FUNCTION "FC_POWER_SAVING_MODE" : VOID
TITLE =POWER SAVING MODE
{ S7_language := '9(1) Angielski (Stany Zjednoczone)  21.09.2015  11:42:42' }
VERSION : 0.1


VAR_TEMP
  CDT : DATE_AND_TIME ;
  READ_CLOCK_RET_VAL : INT ;
  ACT_TIME : TIME_OF_DAY ;
  ACT_TIME_H : INT ;
  ACT_TIME_M : INT ;
  ACT_TIME_S : INT ;
  SW_WD1_ASU_STOP_HEATING : REAL ;
  SW_WD1_ASU_STOP_COOLING : REAL ;
  SW_WD2_ASU_STOP_HEATING : REAL ;
  SW_WD2_ASU_STOP_COOLING : REAL ;
END_VAR
BEGIN
NETWORK
TITLE =READING ACTUAL TIME FROM PLC
//********************************************************************************
//
//                         AUTOMATIC SETPOINTS UPDATE
//
//********************************************************************************
//
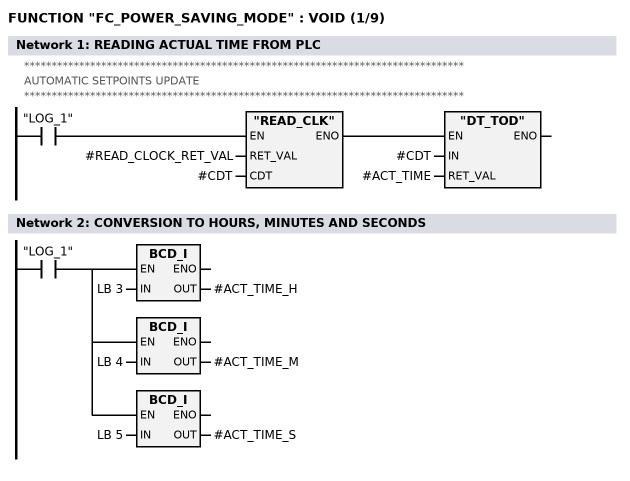
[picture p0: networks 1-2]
      U(    ;
      U     "LOG_1";
      SPBNB _001;
      CALL "READ_CLK" (
           RET_VAL                  := #READ_CLOCK_RET_VAL,
           CDT                      := #CDT);
_001: U     BIE;
      )     ;
      SPBNB _002;
      CALL "DT_TOD" (
           IN                       := #CDT,
           RET_VAL                  := #ACT_TIME);
_002: NOP   0;
NETWORK
TITLE =CONVERSION TO HOURS, MINUTES AND SECONDS

      U     "LOG_1";
      =     L     36.0;
      U     L     36.0;
      SPBNB _003;
      L     LB     3;
      BTI   ;
      T     #ACT_TIME_H;
_003: NOP   0;
      U     L     36.0;
      SPBNB _004;
      L     LB     4;
      BTI   ;
      T     #ACT_TIME_M;
_004: NOP   0;
      U     L     36.0;
      SPBNB _005;
      L     LB     5;
      BTI   ;
      T     #ACT_TIME_S;
_005: NOP   0;
NETWORK
TITLE =LIMIT TIME SET BY OPERATOR
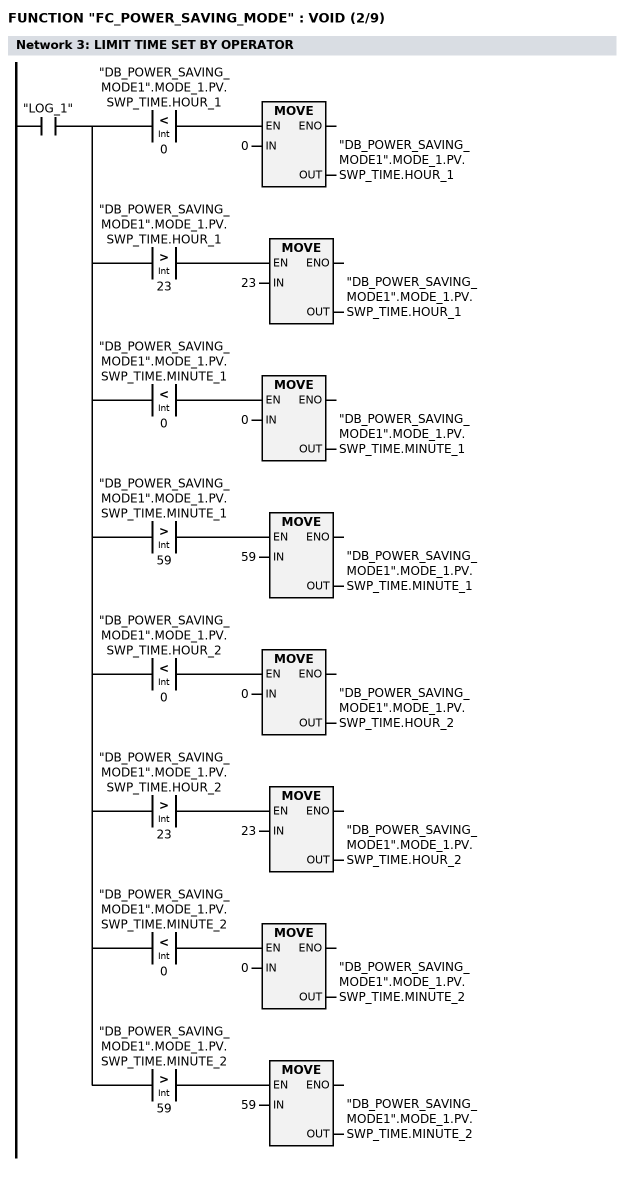
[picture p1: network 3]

      U     "LOG_1";
      =     L     36.0;
      U     L     36.0;
      U(    ;
      L     "DB_POWER_SAVING_MODE1".MODE_1.PV.SWP_TIME.HOUR_1;
      L     0;
      <I    ;
      )     ;
      SPBNB _006;
      L     0;
      T     "DB_POWER_SAVING_MODE1".MODE_1.PV.SWP_TIME.HOUR_1;
_006: NOP   0;
      U     L     36.0;
      U(    ;
      L     "DB_POWER_SAVING_MODE1".MODE_1.PV.SWP_TIME.HOUR_1;
      L     23;
      >I    ;
      )     ;
      SPBNB _007;
      L     23;
      T     "DB_POWER_SAVING_MODE1".MODE_1.PV.SWP_TIME.HOUR_1;
_007: NOP   0;
      U     L     36.0;
      U(    ;
      L     "DB_POWER_SAVING_MODE1".MODE_1.PV.SWP_TIME.MINUTE_1;
      L     0;
      <I    ;
      )     ;
      SPBNB _008;
      L     0;
      T     "DB_POWER_SAVING_MODE1".MODE_1.PV.SWP_TIME.MINUTE_1;
_008: NOP   0;
      U     L     36.0;
      U(    ;
      L     "DB_POWER_SAVING_MODE1".MODE_1.PV.SWP_TIME.MINUTE_1;
      L     59;
      >I    ;
      )     ;
      SPBNB _009;
      L     59;
      T     "DB_POWER_SAVING_MODE1".MODE_1.PV.SWP_TIME.MINUTE_1;
_009: NOP   0;
      U     L     36.0;
      U(    ;
      L     "DB_POWER_SAVING_MODE1".MODE_1.PV.SWP_TIME.HOUR_2;
      L     0;
      <I    ;
      )     ;
      SPBNB _00a;
      L     0;
      T     "DB_POWER_SAVING_MODE1".MODE_1.PV.SWP_TIME.HOUR_2;
_00a: NOP   0;
      U     L     36.0;
      U(    ;
      L     "DB_POWER_SAVING_MODE1".MODE_1.PV.SWP_TIME.HOUR_2;
      L     23;
      >I    ;
      )     ;
      SPBNB _00b;
      L     23;
      T     "DB_POWER_SAVING_MODE1".MODE_1.PV.SWP_TIME.HOUR_2;
_00b: NOP   0;
      U     L     36.0;
      U(    ;
      L     "DB_POWER_SAVING_MODE1".MODE_1.PV.SWP_TIME.MINUTE_2;
      L     0;
      <I    ;
      )     ;
      SPBNB _00c;
      L     0;
      T     "DB_POWER_SAVING_MODE1".MODE_1.PV.SWP_TIME.MINUTE_2;
_00c: NOP   0;
      U     L     36.0;
      U(    ;
      L     "DB_POWER_SAVING_MODE1".MODE_1.PV.SWP_TIME.MINUTE_2;
      L     59;
      >I    ;
      )     ;
      SPBNB _00d;
      L     59;
      T     "DB_POWER_SAVING_MODE1".MODE_1.PV.SWP_TIME.MINUTE_2;
_00d: NOP   0;
NETWORK
TITLE =CHANGE SETPOINTS TWO TIMES PER DAY ACCORDING TO TIME SET
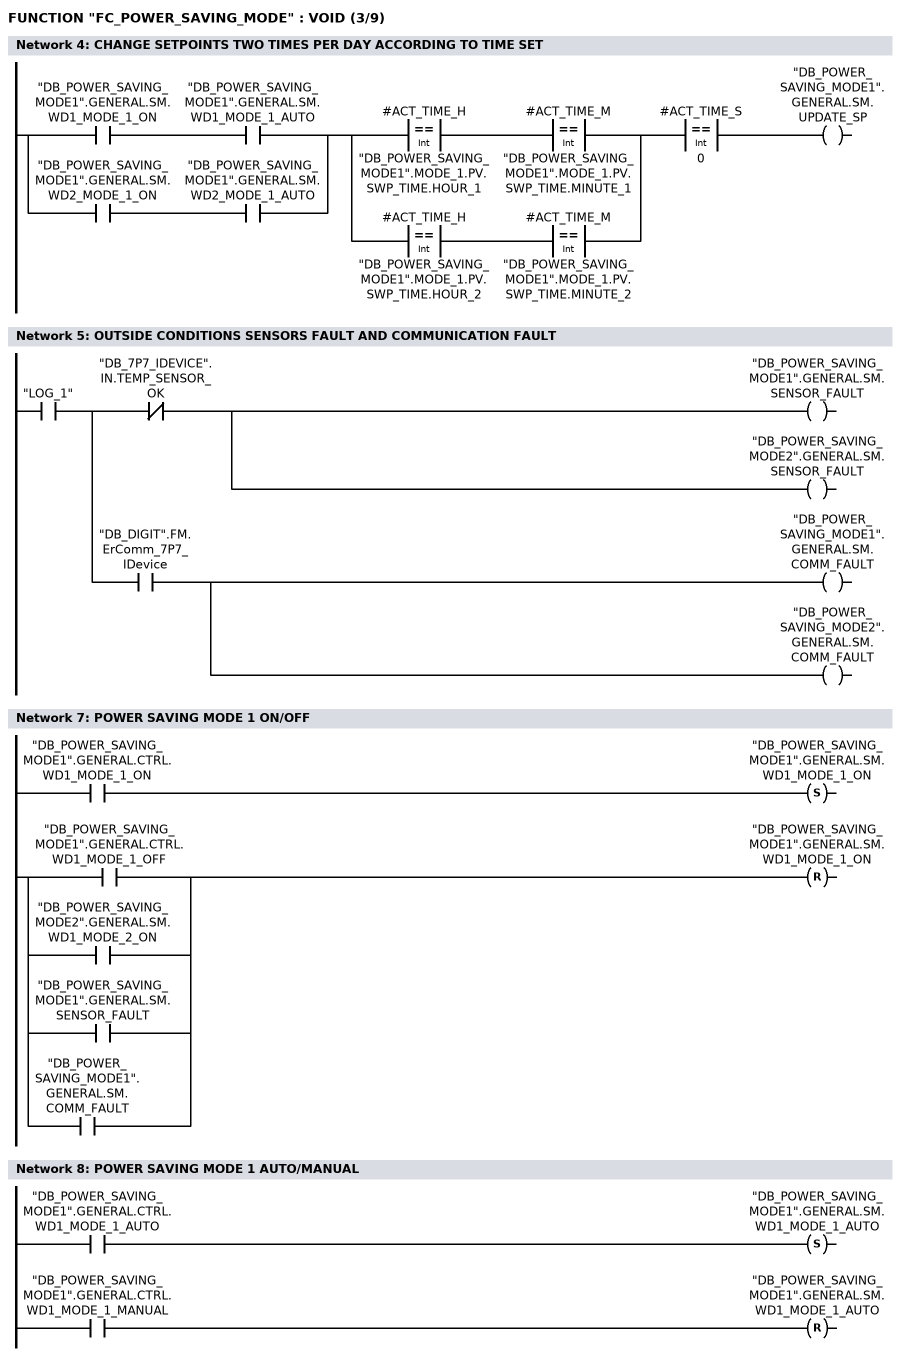
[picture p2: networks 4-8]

      U(    ;
      U     "DB_POWER_SAVING_MODE1".GENERAL.SM.WD1_MODE_1_ON;
      U     "DB_POWER_SAVING_MODE1".GENERAL.SM.WD1_MODE_1_AUTO;
      O     ;
      U     "DB_POWER_SAVING_MODE1".GENERAL.SM.WD2_MODE_1_ON;
      U     "DB_POWER_SAVING_MODE1".GENERAL.SM.WD2_MODE_1_AUTO;
      )     ;
      U(    ;
      U(    ;
      L     #ACT_TIME_H;
      L     "DB_POWER_SAVING_MODE1".MODE_1.PV.SWP_TIME.HOUR_1;
      ==I   ;
      )     ;
      U(    ;
      L     #ACT_TIME_M;
      L     "DB_POWER_SAVING_MODE1".MODE_1.PV.SWP_TIME.MINUTE_1;
      ==I   ;
      )     ;
      O     ;
      U(    ;
      L     #ACT_TIME_H;
      L     "DB_POWER_SAVING_MODE1".MODE_1.PV.SWP_TIME.HOUR_2;
      ==I   ;
      )     ;
      U(    ;
      L     #ACT_TIME_M;
      L     "DB_POWER_SAVING_MODE1".MODE_1.PV.SWP_TIME.MINUTE_2;
      ==I   ;
      )     ;
      )     ;
      U(    ;
      L     #ACT_TIME_S;
      L     0;
      ==I   ;
      )     ;
      =     "DB_POWER_SAVING_MODE1".GENERAL.SM.UPDATE_SP;
NETWORK
TITLE =OUTSIDE CONDITIONS SENSORS FAULT AND COMMUNICATION FAULT

      U     "LOG_1";
      =     L     36.0;
      U     L     36.0;
      UN    "DB_7P7_IDEVICE".IN.TEMP_SENSOR_OK;
      =     "DB_POWER_SAVING_MODE1".GENERAL.SM.SENSOR_FAULT;
      =     "DB_POWER_SAVING_MODE2".GENERAL.SM.SENSOR_FAULT;
      U     L     36.0;
      U     "DB_DIGIT".FM.ErComm_7P7_IDevice;
      =     "DB_POWER_SAVING_MODE1".GENERAL.SM.COMM_FAULT;
      =     "DB_POWER_SAVING_MODE2".GENERAL.SM.COMM_FAULT;
NETWORK
TITLE =********* WORKDECK'S 1 ECO MODE 1 **************
//********************************************************************************
//
//                     WORKDECK'S 1 POWER SAVING MODE 1
//
//********************************************************************************
//
NETWORK
TITLE =POWER SAVING MODE 1 ON/OFF

      U     "DB_POWER_SAVING_MODE1".GENERAL.CTRL.WD1_MODE_1_ON;
      S     "DB_POWER_SAVING_MODE1".GENERAL.SM.WD1_MODE_1_ON;
      U(    ;
      O     "DB_POWER_SAVING_MODE1".GENERAL.CTRL.WD1_MODE_1_OFF;
      O     "DB_POWER_SAVING_MODE2".GENERAL.SM.WD1_MODE_2_ON;
      O     "DB_POWER_SAVING_MODE1".GENERAL.SM.SENSOR_FAULT;
      O     "DB_POWER_SAVING_MODE1".GENERAL.SM.COMM_FAULT;
      )     ;
      R     "DB_POWER_SAVING_MODE1".GENERAL.SM.WD1_MODE_1_ON;
      NOP   0;
NETWORK
TITLE =POWER SAVING MODE 1 AUTO/MANUAL

      U     "DB_POWER_SAVING_MODE1".GENERAL.CTRL.WD1_MODE_1_AUTO;
      S     "DB_POWER_SAVING_MODE1".GENERAL.SM.WD1_MODE_1_AUTO;
      U     "DB_POWER_SAVING_MODE1".GENERAL.CTRL.WD1_MODE_1_MANUAL;
      R     "DB_POWER_SAVING_MODE1".GENERAL.SM.WD1_MODE_1_AUTO;
      NOP   0;
NETWORK
TITLE =
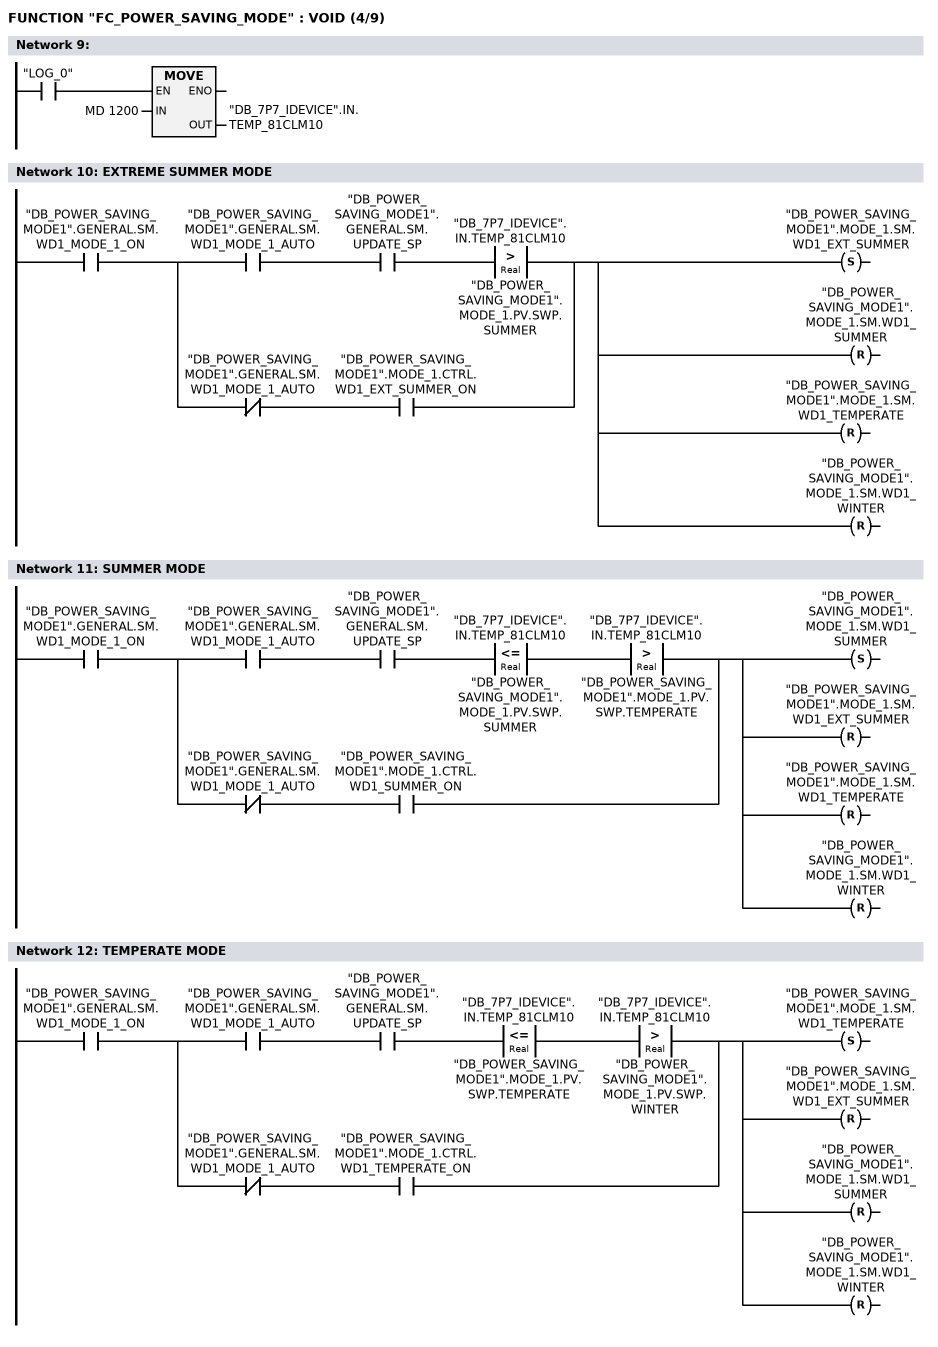
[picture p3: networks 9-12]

      U     "LOG_0";
      SPBNB _00e;
      L     MD  1200;
      T     "DB_7P7_IDEVICE".IN.TEMP_81CLM10;
_00e: NOP   0;
NETWORK
TITLE =EXTREME SUMMER MODE

      U     "DB_POWER_SAVING_MODE1".GENERAL.SM.WD1_MODE_1_ON;
      U(    ;
      U     "DB_POWER_SAVING_MODE1".GENERAL.SM.WD1_MODE_1_AUTO;
      U     "DB_POWER_SAVING_MODE1".GENERAL.SM.UPDATE_SP;
      U(    ;
      L     "DB_7P7_IDEVICE".IN.TEMP_81CLM10;
      L     "DB_POWER_SAVING_MODE1".MODE_1.PV.SWP.SUMMER;
      >R    ;
      )     ;
      O     ;
      UN    "DB_POWER_SAVING_MODE1".GENERAL.SM.WD1_MODE_1_AUTO;
      U     "DB_POWER_SAVING_MODE1".MODE_1.CTRL.WD1_EXT_SUMMER_ON;
      )     ;
      S     "DB_POWER_SAVING_MODE1".MODE_1.SM.WD1_EXT_SUMMER;
      R     "DB_POWER_SAVING_MODE1".MODE_1.SM.WD1_SUMMER;
      R     "DB_POWER_SAVING_MODE1".MODE_1.SM.WD1_TEMPERATE;
      R     "DB_POWER_SAVING_MODE1".MODE_1.SM.WD1_WINTER;
NETWORK
TITLE =SUMMER MODE

      U     "DB_POWER_SAVING_MODE1".GENERAL.SM.WD1_MODE_1_ON;
      U(    ;
      U     "DB_POWER_SAVING_MODE1".GENERAL.SM.WD1_MODE_1_AUTO;
      U     "DB_POWER_SAVING_MODE1".GENERAL.SM.UPDATE_SP;
      U(    ;
      L     "DB_7P7_IDEVICE".IN.TEMP_81CLM10;
      L     "DB_POWER_SAVING_MODE1".MODE_1.PV.SWP.SUMMER;
      <=R   ;
      )     ;
      U(    ;
      L     "DB_7P7_IDEVICE".IN.TEMP_81CLM10;
      L     "DB_POWER_SAVING_MODE1".MODE_1.PV.SWP.TEMPERATE;
      >R    ;
      )     ;
      O     ;
      UN    "DB_POWER_SAVING_MODE1".GENERAL.SM.WD1_MODE_1_AUTO;
      U     "DB_POWER_SAVING_MODE1".MODE_1.CTRL.WD1_SUMMER_ON;
      )     ;
      S     "DB_POWER_SAVING_MODE1".MODE_1.SM.WD1_SUMMER;
      R     "DB_POWER_SAVING_MODE1".MODE_1.SM.WD1_EXT_SUMMER;
      R     "DB_POWER_SAVING_MODE1".MODE_1.SM.WD1_TEMPERATE;
      R     "DB_POWER_SAVING_MODE1".MODE_1.SM.WD1_WINTER;
NETWORK
TITLE =TEMPERATE MODE

      U     "DB_POWER_SAVING_MODE1".GENERAL.SM.WD1_MODE_1_ON;
      U(    ;
      U     "DB_POWER_SAVING_MODE1".GENERAL.SM.WD1_MODE_1_AUTO;
      U     "DB_POWER_SAVING_MODE1".GENERAL.SM.UPDATE_SP;
      U(    ;
      L     "DB_7P7_IDEVICE".IN.TEMP_81CLM10;
      L     "DB_POWER_SAVING_MODE1".MODE_1.PV.SWP.TEMPERATE;
      <=R   ;
      )     ;
      U(    ;
      L     "DB_7P7_IDEVICE".IN.TEMP_81CLM10;
      L     "DB_POWER_SAVING_MODE1".MODE_1.PV.SWP.WINTER;
      >R    ;
      )     ;
      O     ;
      UN    "DB_POWER_SAVING_MODE1".GENERAL.SM.WD1_MODE_1_AUTO;
      U     "DB_POWER_SAVING_MODE1".MODE_1.CTRL.WD1_TEMPERATE_ON;
      )     ;
      S     "DB_POWER_SAVING_MODE1".MODE_1.SM.WD1_TEMPERATE;
      R     "DB_POWER_SAVING_MODE1".MODE_1.SM.WD1_EXT_SUMMER;
      R     "DB_POWER_SAVING_MODE1".MODE_1.SM.WD1_SUMMER;
      R     "DB_POWER_SAVING_MODE1".MODE_1.SM.WD1_WINTER;
NETWORK
TITLE =WINTER MODE
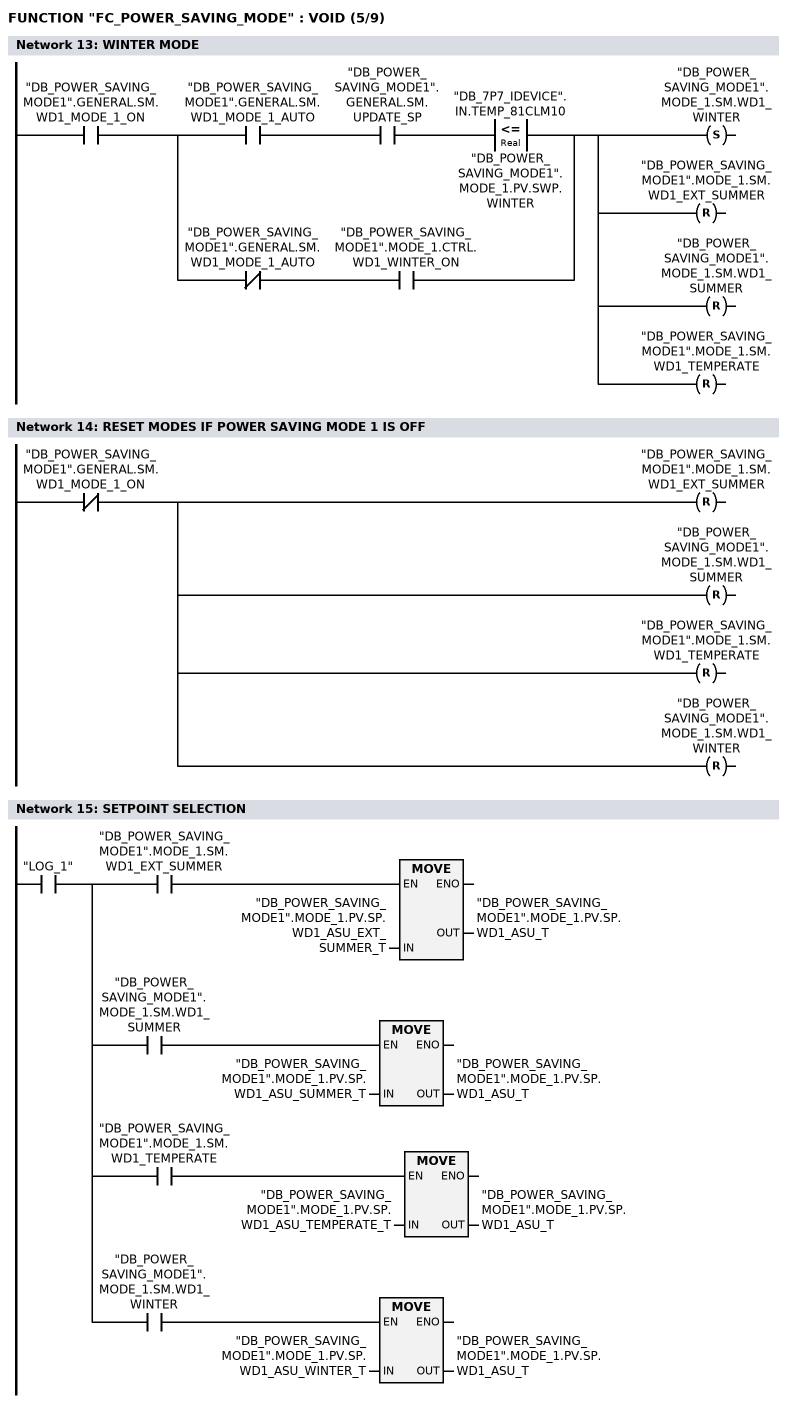
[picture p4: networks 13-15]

      U     "DB_POWER_SAVING_MODE1".GENERAL.SM.WD1_MODE_1_ON;
      U(    ;
      U     "DB_POWER_SAVING_MODE1".GENERAL.SM.WD1_MODE_1_AUTO;
      U     "DB_POWER_SAVING_MODE1".GENERAL.SM.UPDATE_SP;
      U(    ;
      L     "DB_7P7_IDEVICE".IN.TEMP_81CLM10;
      L     "DB_POWER_SAVING_MODE1".MODE_1.PV.SWP.WINTER;
      <=R   ;
      )     ;
      O     ;
      UN    "DB_POWER_SAVING_MODE1".GENERAL.SM.WD1_MODE_1_AUTO;
      U     "DB_POWER_SAVING_MODE1".MODE_1.CTRL.WD1_WINTER_ON;
      )     ;
      S     "DB_POWER_SAVING_MODE1".MODE_1.SM.WD1_WINTER;
      R     "DB_POWER_SAVING_MODE1".MODE_1.SM.WD1_EXT_SUMMER;
      R     "DB_POWER_SAVING_MODE1".MODE_1.SM.WD1_SUMMER;
      R     "DB_POWER_SAVING_MODE1".MODE_1.SM.WD1_TEMPERATE;
NETWORK
TITLE =RESET MODES IF POWER SAVING MODE 1 IS OFF

      UN    "DB_POWER_SAVING_MODE1".GENERAL.SM.WD1_MODE_1_ON;
      R     "DB_POWER_SAVING_MODE1".MODE_1.SM.WD1_EXT_SUMMER;
      R     "DB_POWER_SAVING_MODE1".MODE_1.SM.WD1_SUMMER;
      R     "DB_POWER_SAVING_MODE1".MODE_1.SM.WD1_TEMPERATE;
      R     "DB_POWER_SAVING_MODE1".MODE_1.SM.WD1_WINTER;
NETWORK
TITLE =SETPOINT SELECTION

      U     "LOG_1";
      =     L     36.0;
      U     L     36.0;
      U     "DB_POWER_SAVING_MODE1".MODE_1.SM.WD1_EXT_SUMMER;
      SPBNB _00f;
      L     "DB_POWER_SAVING_MODE1".MODE_1.PV.SP.WD1_ASU_EXT_SUMMER_T;
      T     "DB_POWER_SAVING_MODE1".MODE_1.PV.SP.WD1_ASU_T;
_00f: NOP   0;
      U     L     36.0;
      U     "DB_POWER_SAVING_MODE1".MODE_1.SM.WD1_SUMMER;
      SPBNB _010;
      L     "DB_POWER_SAVING_MODE1".MODE_1.PV.SP.WD1_ASU_SUMMER_T;
      T     "DB_POWER_SAVING_MODE1".MODE_1.PV.SP.WD1_ASU_T;
_010: NOP   0;
      U     L     36.0;
      U     "DB_POWER_SAVING_MODE1".MODE_1.SM.WD1_TEMPERATE;
      SPBNB _011;
      L     "DB_POWER_SAVING_MODE1".MODE_1.PV.SP.WD1_ASU_TEMPERATE_T;
      T     "DB_POWER_SAVING_MODE1".MODE_1.PV.SP.WD1_ASU_T;
_011: NOP   0;
      U     L     36.0;
      U     "DB_POWER_SAVING_MODE1".MODE_1.SM.WD1_WINTER;
      SPBNB _012;
      L     "DB_POWER_SAVING_MODE1".MODE_1.PV.SP.WD1_ASU_WINTER_T;
      T     "DB_POWER_SAVING_MODE1".MODE_1.PV.SP.WD1_ASU_T;
_012: NOP   0;
NETWORK
TITLE =DEFAULT MODE - TEMPERATE
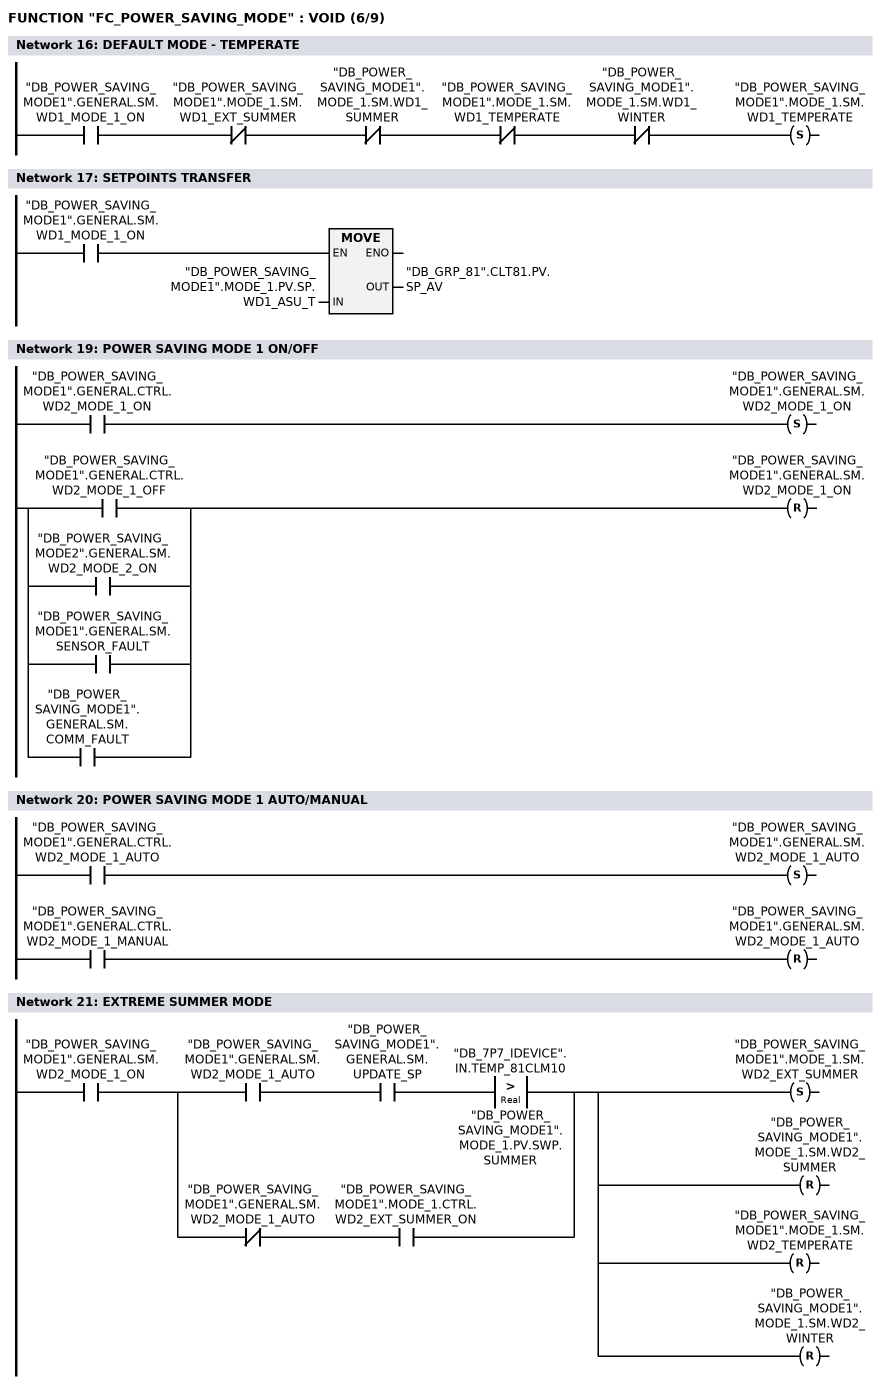
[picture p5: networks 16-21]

      U     "DB_POWER_SAVING_MODE1".GENERAL.SM.WD1_MODE_1_ON;
      UN    "DB_POWER_SAVING_MODE1".MODE_1.SM.WD1_EXT_SUMMER;
      UN    "DB_POWER_SAVING_MODE1".MODE_1.SM.WD1_SUMMER;
      UN    "DB_POWER_SAVING_MODE1".MODE_1.SM.WD1_TEMPERATE;
      UN    "DB_POWER_SAVING_MODE1".MODE_1.SM.WD1_WINTER;
      S     "DB_POWER_SAVING_MODE1".MODE_1.SM.WD1_TEMPERATE;
NETWORK
TITLE =SETPOINTS TRANSFER

      U     "DB_POWER_SAVING_MODE1".GENERAL.SM.WD1_MODE_1_ON;
      SPBNB _013;
      L     "DB_POWER_SAVING_MODE1".MODE_1.PV.SP.WD1_ASU_T;
      T     "DB_GRP_81".CLT81.PV.SP_AV;
_013: NOP   0;
NETWORK
TITLE =************ WORKDECK'S 2 ECO MODE 1 ***********
//********************************************************************************
//
//                        WORKDECK'S 2 POWER SAVING MODE 1
//
//********************************************************************************
//
NETWORK
TITLE =POWER SAVING MODE 1 ON/OFF

      U     "DB_POWER_SAVING_MODE1".GENERAL.CTRL.WD2_MODE_1_ON;
      S     "DB_POWER_SAVING_MODE1".GENERAL.SM.WD2_MODE_1_ON;
      U(    ;
      O     "DB_POWER_SAVING_MODE1".GENERAL.CTRL.WD2_MODE_1_OFF;
      O     "DB_POWER_SAVING_MODE2".GENERAL.SM.WD2_MODE_2_ON;
      O     "DB_POWER_SAVING_MODE1".GENERAL.SM.SENSOR_FAULT;
      O     "DB_POWER_SAVING_MODE1".GENERAL.SM.COMM_FAULT;
      )     ;
      R     "DB_POWER_SAVING_MODE1".GENERAL.SM.WD2_MODE_1_ON;
      NOP   0;
NETWORK
TITLE =POWER SAVING MODE 1 AUTO/MANUAL

      U     "DB_POWER_SAVING_MODE1".GENERAL.CTRL.WD2_MODE_1_AUTO;
      S     "DB_POWER_SAVING_MODE1".GENERAL.SM.WD2_MODE_1_AUTO;
      U     "DB_POWER_SAVING_MODE1".GENERAL.CTRL.WD2_MODE_1_MANUAL;
      R     "DB_POWER_SAVING_MODE1".GENERAL.SM.WD2_MODE_1_AUTO;
      NOP   0;
NETWORK
TITLE =EXTREME SUMMER MODE

      U     "DB_POWER_SAVING_MODE1".GENERAL.SM.WD2_MODE_1_ON;
      U(    ;
      U     "DB_POWER_SAVING_MODE1".GENERAL.SM.WD2_MODE_1_AUTO;
      U     "DB_POWER_SAVING_MODE1".GENERAL.SM.UPDATE_SP;
      U(    ;
      L     "DB_7P7_IDEVICE".IN.TEMP_81CLM10;
      L     "DB_POWER_SAVING_MODE1".MODE_1.PV.SWP.SUMMER;
      >R    ;
      )     ;
      O     ;
      UN    "DB_POWER_SAVING_MODE1".GENERAL.SM.WD2_MODE_1_AUTO;
      U     "DB_POWER_SAVING_MODE1".MODE_1.CTRL.WD2_EXT_SUMMER_ON;
      )     ;
      S     "DB_POWER_SAVING_MODE1".MODE_1.SM.WD2_EXT_SUMMER;
      R     "DB_POWER_SAVING_MODE1".MODE_1.SM.WD2_SUMMER;
      R     "DB_POWER_SAVING_MODE1".MODE_1.SM.WD2_TEMPERATE;
      R     "DB_POWER_SAVING_MODE1".MODE_1.SM.WD2_WINTER;
NETWORK
TITLE =SUMMER MODE
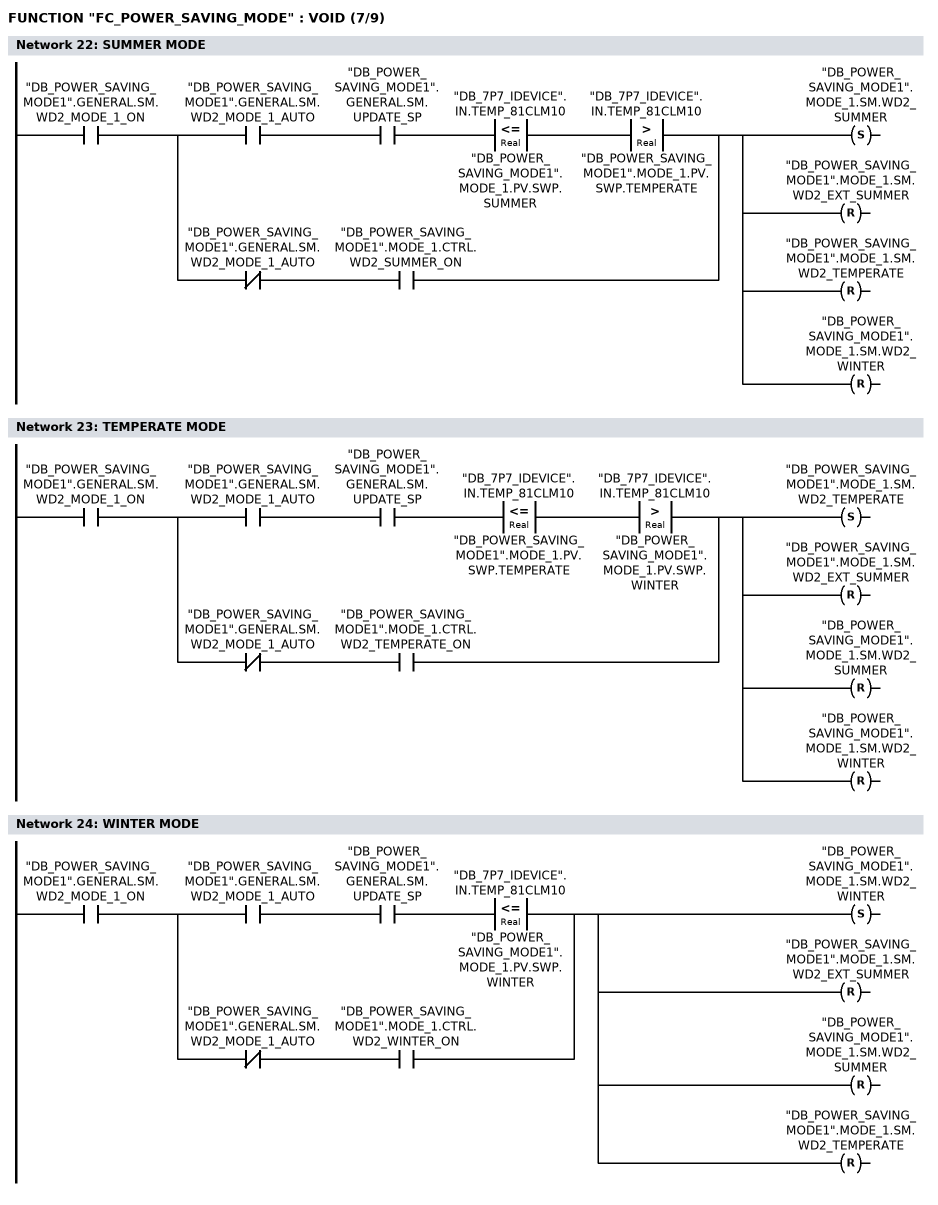
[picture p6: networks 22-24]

      U     "DB_POWER_SAVING_MODE1".GENERAL.SM.WD2_MODE_1_ON;
      U(    ;
      U     "DB_POWER_SAVING_MODE1".GENERAL.SM.WD2_MODE_1_AUTO;
      U     "DB_POWER_SAVING_MODE1".GENERAL.SM.UPDATE_SP;
      U(    ;
      L     "DB_7P7_IDEVICE".IN.TEMP_81CLM10;
      L     "DB_POWER_SAVING_MODE1".MODE_1.PV.SWP.SUMMER;
      <=R   ;
      )     ;
      U(    ;
      L     "DB_7P7_IDEVICE".IN.TEMP_81CLM10;
      L     "DB_POWER_SAVING_MODE1".MODE_1.PV.SWP.TEMPERATE;
      >R    ;
      )     ;
      O     ;
      UN    "DB_POWER_SAVING_MODE1".GENERAL.SM.WD2_MODE_1_AUTO;
      U     "DB_POWER_SAVING_MODE1".MODE_1.CTRL.WD2_SUMMER_ON;
      )     ;
      S     "DB_POWER_SAVING_MODE1".MODE_1.SM.WD2_SUMMER;
      R     "DB_POWER_SAVING_MODE1".MODE_1.SM.WD2_EXT_SUMMER;
      R     "DB_POWER_SAVING_MODE1".MODE_1.SM.WD2_TEMPERATE;
      R     "DB_POWER_SAVING_MODE1".MODE_1.SM.WD2_WINTER;
NETWORK
TITLE =TEMPERATE MODE

      U     "DB_POWER_SAVING_MODE1".GENERAL.SM.WD2_MODE_1_ON;
      U(    ;
      U     "DB_POWER_SAVING_MODE1".GENERAL.SM.WD2_MODE_1_AUTO;
      U     "DB_POWER_SAVING_MODE1".GENERAL.SM.UPDATE_SP;
      U(    ;
      L     "DB_7P7_IDEVICE".IN.TEMP_81CLM10;
      L     "DB_POWER_SAVING_MODE1".MODE_1.PV.SWP.TEMPERATE;
      <=R   ;
      )     ;
      U(    ;
      L     "DB_7P7_IDEVICE".IN.TEMP_81CLM10;
      L     "DB_POWER_SAVING_MODE1".MODE_1.PV.SWP.WINTER;
      >R    ;
      )     ;
      O     ;
      UN    "DB_POWER_SAVING_MODE1".GENERAL.SM.WD2_MODE_1_AUTO;
      U     "DB_POWER_SAVING_MODE1".MODE_1.CTRL.WD2_TEMPERATE_ON;
      )     ;
      S     "DB_POWER_SAVING_MODE1".MODE_1.SM.WD2_TEMPERATE;
      R     "DB_POWER_SAVING_MODE1".MODE_1.SM.WD2_EXT_SUMMER;
      R     "DB_POWER_SAVING_MODE1".MODE_1.SM.WD2_SUMMER;
      R     "DB_POWER_SAVING_MODE1".MODE_1.SM.WD2_WINTER;
NETWORK
TITLE =WINTER MODE

      U     "DB_POWER_SAVING_MODE1".GENERAL.SM.WD2_MODE_1_ON;
      U(    ;
      U     "DB_POWER_SAVING_MODE1".GENERAL.SM.WD2_MODE_1_AUTO;
      U     "DB_POWER_SAVING_MODE1".GENERAL.SM.UPDATE_SP;
      U(    ;
      L     "DB_7P7_IDEVICE".IN.TEMP_81CLM10;
      L     "DB_POWER_SAVING_MODE1".MODE_1.PV.SWP.WINTER;
      <=R   ;
      )     ;
      O     ;
      UN    "DB_POWER_SAVING_MODE1".GENERAL.SM.WD2_MODE_1_AUTO;
      U     "DB_POWER_SAVING_MODE1".MODE_1.CTRL.WD2_WINTER_ON;
      )     ;
      S     "DB_POWER_SAVING_MODE1".MODE_1.SM.WD2_WINTER;
      R     "DB_POWER_SAVING_MODE1".MODE_1.SM.WD2_EXT_SUMMER;
      R     "DB_POWER_SAVING_MODE1".MODE_1.SM.WD2_SUMMER;
      R     "DB_POWER_SAVING_MODE1".MODE_1.SM.WD2_TEMPERATE;
NETWORK
TITLE =RESET MODES IF POWER SAVING MODE 1 IS OFF
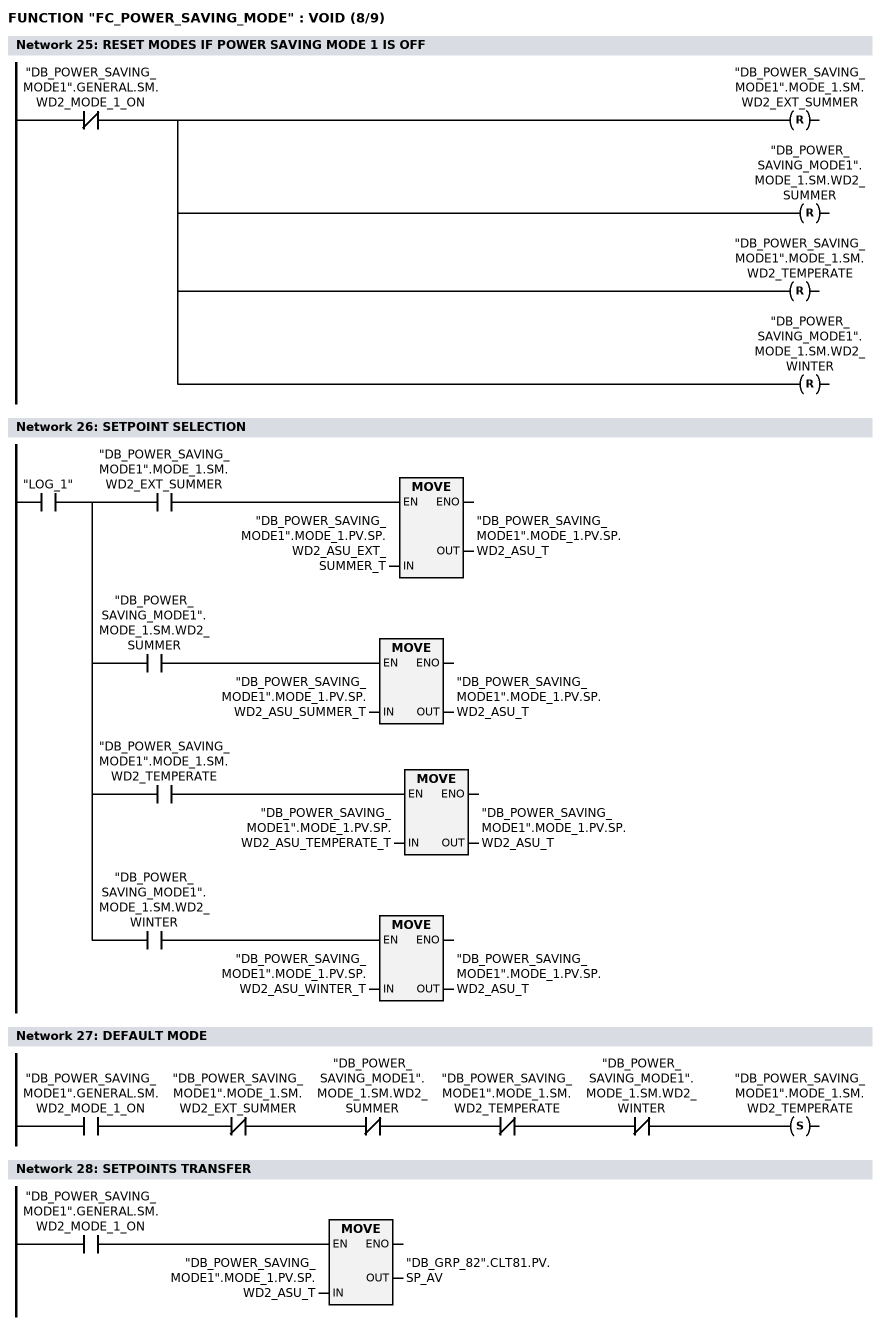
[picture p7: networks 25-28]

      UN    "DB_POWER_SAVING_MODE1".GENERAL.SM.WD2_MODE_1_ON;
      R     "DB_POWER_SAVING_MODE1".MODE_1.SM.WD2_EXT_SUMMER;
      R     "DB_POWER_SAVING_MODE1".MODE_1.SM.WD2_SUMMER;
      R     "DB_POWER_SAVING_MODE1".MODE_1.SM.WD2_TEMPERATE;
      R     "DB_POWER_SAVING_MODE1".MODE_1.SM.WD2_WINTER;
NETWORK
TITLE =SETPOINT SELECTION

      U     "LOG_1";
      =     L     36.0;
      U     L     36.0;
      U     "DB_POWER_SAVING_MODE1".MODE_1.SM.WD2_EXT_SUMMER;
      SPBNB _014;
      L     "DB_POWER_SAVING_MODE1".MODE_1.PV.SP.WD2_ASU_EXT_SUMMER_T;
      T     "DB_POWER_SAVING_MODE1".MODE_1.PV.SP.WD2_ASU_T;
_014: NOP   0;
      U     L     36.0;
      U     "DB_POWER_SAVING_MODE1".MODE_1.SM.WD2_SUMMER;
      SPBNB _015;
      L     "DB_POWER_SAVING_MODE1".MODE_1.PV.SP.WD2_ASU_SUMMER_T;
      T     "DB_POWER_SAVING_MODE1".MODE_1.PV.SP.WD2_ASU_T;
_015: NOP   0;
      U     L     36.0;
      U     "DB_POWER_SAVING_MODE1".MODE_1.SM.WD2_TEMPERATE;
      SPBNB _016;
      L     "DB_POWER_SAVING_MODE1".MODE_1.PV.SP.WD2_ASU_TEMPERATE_T;
      T     "DB_POWER_SAVING_MODE1".MODE_1.PV.SP.WD2_ASU_T;
_016: NOP   0;
      U     L     36.0;
      U     "DB_POWER_SAVING_MODE1".MODE_1.SM.WD2_WINTER;
      SPBNB _017;
      L     "DB_POWER_SAVING_MODE1".MODE_1.PV.SP.WD2_ASU_WINTER_T;
      T     "DB_POWER_SAVING_MODE1".MODE_1.PV.SP.WD2_ASU_T;
_017: NOP   0;
NETWORK
TITLE =DEFAULT MODE

      U     "DB_POWER_SAVING_MODE1".GENERAL.SM.WD2_MODE_1_ON;
      UN    "DB_POWER_SAVING_MODE1".MODE_1.SM.WD2_EXT_SUMMER;
      UN    "DB_POWER_SAVING_MODE1".MODE_1.SM.WD2_SUMMER;
      UN    "DB_POWER_SAVING_MODE1".MODE_1.SM.WD2_TEMPERATE;
      UN    "DB_POWER_SAVING_MODE1".MODE_1.SM.WD2_WINTER;
      S     "DB_POWER_SAVING_MODE1".MODE_1.SM.WD2_TEMPERATE;
NETWORK
TITLE =SETPOINTS TRANSFER

      U     "DB_POWER_SAVING_MODE1".GENERAL.SM.WD2_MODE_1_ON;
      SPBNB _018;
      L     "DB_POWER_SAVING_MODE1".MODE_1.PV.SP.WD2_ASU_T;
      T     "DB_GRP_82".CLT81.PV.SP_AV;
_018: NOP   0;
NETWORK
TITLE =************* WORKDECK'S 1/2 ECO MODE 2 ************
//********************************************************************************
//
//                     WORKDECK'S 1/2 POWER SAVING MODE 2
//
//********************************************************************************
//
NETWORK
TITLE =POWER SAVING MODE 2 WORKDECK'S 1 ON/OFF
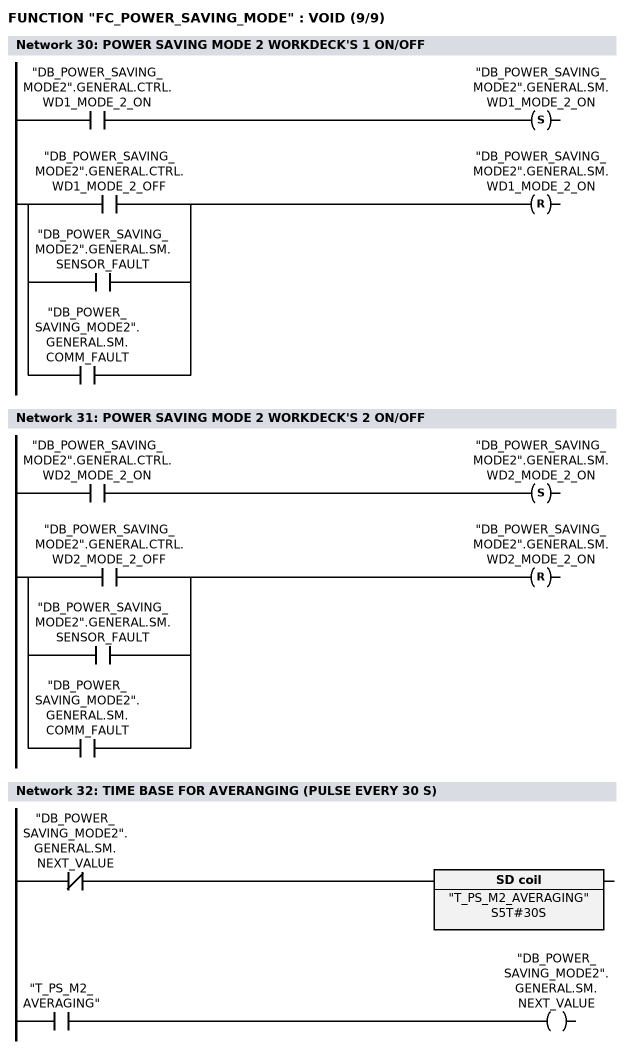
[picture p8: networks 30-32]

      U     "DB_POWER_SAVING_MODE2".GENERAL.CTRL.WD1_MODE_2_ON;
      S     "DB_POWER_SAVING_MODE2".GENERAL.SM.WD1_MODE_2_ON;
      U(    ;
      O     "DB_POWER_SAVING_MODE2".GENERAL.CTRL.WD1_MODE_2_OFF;
      O     "DB_POWER_SAVING_MODE2".GENERAL.SM.SENSOR_FAULT;
      O     "DB_POWER_SAVING_MODE2".GENERAL.SM.COMM_FAULT;
      )     ;
      R     "DB_POWER_SAVING_MODE2".GENERAL.SM.WD1_MODE_2_ON;
      NOP   0;
NETWORK
TITLE =POWER SAVING MODE 2 WORKDECK'S 2 ON/OFF

      U     "DB_POWER_SAVING_MODE2".GENERAL.CTRL.WD2_MODE_2_ON;
      S     "DB_POWER_SAVING_MODE2".GENERAL.SM.WD2_MODE_2_ON;
      U(    ;
      O     "DB_POWER_SAVING_MODE2".GENERAL.CTRL.WD2_MODE_2_OFF;
      O     "DB_POWER_SAVING_MODE2".GENERAL.SM.SENSOR_FAULT;
      O     "DB_POWER_SAVING_MODE2".GENERAL.SM.COMM_FAULT;
      )     ;
      R     "DB_POWER_SAVING_MODE2".GENERAL.SM.WD2_MODE_2_ON;
      NOP   0;
NETWORK
TITLE =TIME BASE FOR AVERANGING (PULSE EVERY 30 S)

      UN    "DB_POWER_SAVING_MODE2".GENERAL.SM.NEXT_VALUE;
      L     S5T#30S;
      SE    "T_PS_M2_AVERAGING";

      U     "T_PS_M2_AVERAGING";
      =     "DB_POWER_SAVING_MODE2".GENERAL.SM.NEXT_VALUE;

NETWORK
TITLE =10 MIN AVERAGE OF OUTSIDE TEMPERATURE

      UN    "DB_POWER_SAVING_MODE2".GENERAL.SM.SENSOR_FAULT;
      =     L     36.0;
      U     "DB_POWER_SAVING_MODE2".GENERAL.SM.NEXT_VALUE;
      =     L     36.1;
      BLD   103;
      U     L     36.0;
      SPBNB _019;
      CALL "FB_AVERAGING" , "DBI_81CLM10_TEMP_AVR" (
           IiNumberOfAddend         := 20,
           IrMeasuringValue         := "DB_7P7_IDEVICE".IN.TEMP_81CLM10,
           IxNewValueAvailable      := L     36.1);

_019: NOP   0;
      U     L     36.0;
      SPBNB _01a;
      L     "DBI_81CLM10_TEMP_AVR".QrAverageValue;
      T     "DB_POWER_SAVING_MODE2".GENERAL.PV.AVG_TEMP;
_01a: NOP   0;
NETWORK
TITLE =************** START ECO MODE 2 WORKDECK'S 1 *************

NETWORK
TITLE =WORKDECK'S 1 ASU OUTSIDE CONDITIONS
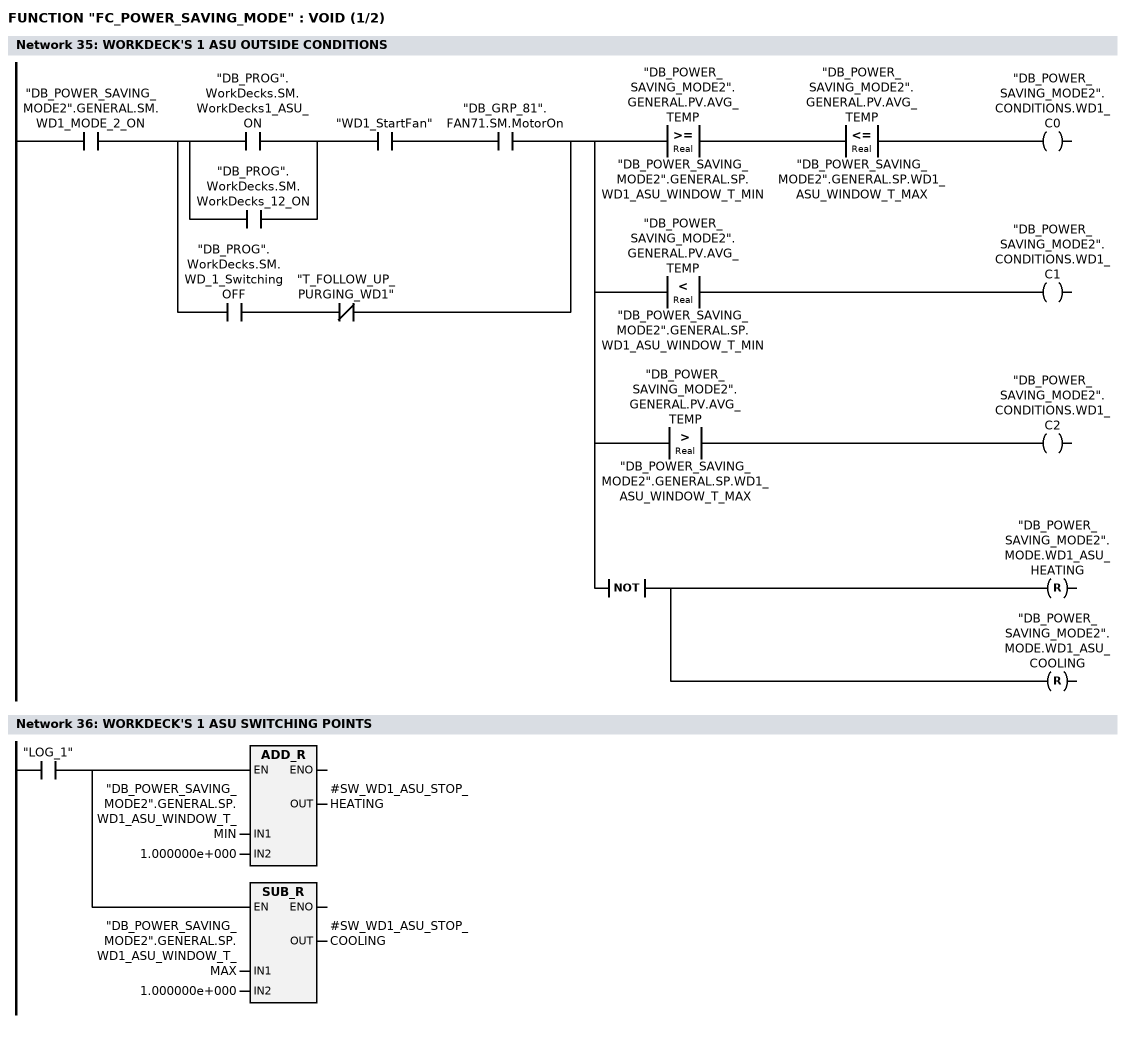
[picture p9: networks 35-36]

      U     "DB_POWER_SAVING_MODE2".GENERAL.SM.WD1_MODE_2_ON;
      U(    ;
      U(    ;
      O     "DB_PROG".WorkDecks.SM.WorkDecks1_ASU_ON;
      O     "DB_PROG".WorkDecks.SM.WorkDecks_12_ON;
      )     ;
      U     "WD1_StartFan";
      U     "DB_GRP_81".FAN71.SM.MotorOn;
      O     ;
      U     "DB_PROG".WorkDecks.SM.WD_1_SwitchingOFF;
      UN    "T_FOLLOW_UP_PURGING_WD1";
      )     ;
      =     L     36.0;
      U     L     36.0;
      U(    ;
      L     "DB_POWER_SAVING_MODE2".GENERAL.PV.AVG_TEMP;
      L     "DB_POWER_SAVING_MODE2".GENERAL.SP.WD1_ASU_WINDOW_T_MIN;
      >=R   ;
      )     ;
      U(    ;
      L     "DB_POWER_SAVING_MODE2".GENERAL.PV.AVG_TEMP;
      L     "DB_POWER_SAVING_MODE2".GENERAL.SP.WD1_ASU_WINDOW_T_MAX;
      <=R   ;
      )     ;
      =     "DB_POWER_SAVING_MODE2".CONDITIONS.WD1_C0;
      U     L     36.0;
      U(    ;
      L     "DB_POWER_SAVING_MODE2".GENERAL.PV.AVG_TEMP;
      L     "DB_POWER_SAVING_MODE2".GENERAL.SP.WD1_ASU_WINDOW_T_MIN;
      <R    ;
      )     ;
      =     "DB_POWER_SAVING_MODE2".CONDITIONS.WD1_C1;
      U     L     36.0;
      U(    ;
      L     "DB_POWER_SAVING_MODE2".GENERAL.PV.AVG_TEMP;
      L     "DB_POWER_SAVING_MODE2".GENERAL.SP.WD1_ASU_WINDOW_T_MAX;
      >R    ;
      )     ;
      =     "DB_POWER_SAVING_MODE2".CONDITIONS.WD1_C2;
      U     L     36.0;
      NOT   ;
      R     "DB_POWER_SAVING_MODE2".MODE.WD1_ASU_HEATING;
      R     "DB_POWER_SAVING_MODE2".MODE.WD1_ASU_COOLING;
NETWORK
TITLE =WORKDECK'S 1 ASU SWITCHING POINTS

      U     "LOG_1";
      =     L     36.0;
      U     L     36.0;
      SPBNB _01b;
      L     "DB_POWER_SAVING_MODE2".GENERAL.SP.WD1_ASU_WINDOW_T_MIN;
      L     1.000000e+000;
      +R    ;
      T     #SW_WD1_ASU_STOP_HEATING;
_01b: NOP   0;
      U     L     36.0;
      SPBNB _01c;
      L     "DB_POWER_SAVING_MODE2".GENERAL.SP.WD1_ASU_WINDOW_T_MAX;
      L     1.000000e+000;
      -R    ;
      T     #SW_WD1_ASU_STOP_COOLING;
_01c: NOP   0;
NETWORK
TITLE =WORKDECK'S 1 CONDIDITON 0
//OUTSIDE TEMPERATURE IN WINDOW
//
//HEATING OFF
//COOLING OFF
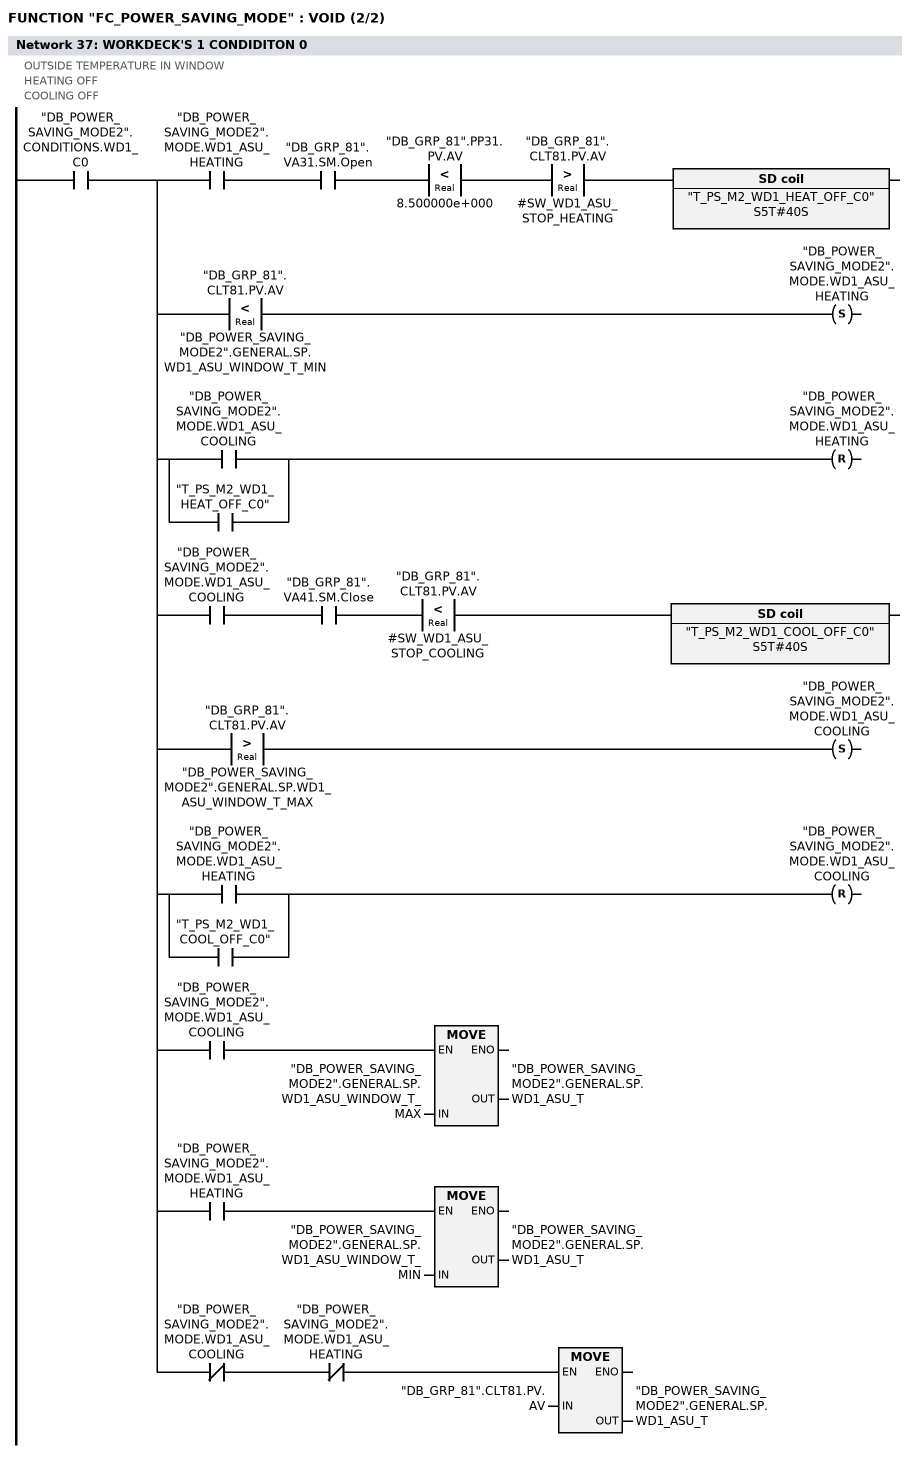
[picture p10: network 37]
      U     "DB_POWER_SAVING_MODE2".CONDITIONS.WD1_C0;
      =     L     36.0;
      U     L     36.0;
      U     "DB_POWER_SAVING_MODE2".MODE.WD1_ASU_HEATING;
      U     "DB_GRP_81".VA31.SM.Open;
      U(    ;
      L     "DB_GRP_81".PP31.PV.AV;
      L     8.500000e+000;
      <R    ;
      )     ;
      U(    ;
      L     "DB_GRP_81".CLT81.PV.AV;
      L     #SW_WD1_ASU_STOP_HEATING;
      >R    ;
      )     ;
      L     S5T#40S;
      SE    "T_PS_M2_WD1_HEAT_OFF_C0";
      NOP   0;
      NOP   0;
      NOP   0;
      NOP   0;
      U     L     36.0;
      U(    ;
      L     "DB_GRP_81".CLT81.PV.AV;
      L     "DB_POWER_SAVING_MODE2".GENERAL.SP.WD1_ASU_WINDOW_T_MIN;
      <R    ;
      )     ;
      S     "DB_POWER_SAVING_MODE2".MODE.WD1_ASU_HEATING;
      U     L     36.0;
      U(    ;
      O     "DB_POWER_SAVING_MODE2".MODE.WD1_ASU_COOLING;
      O     "T_PS_M2_WD1_HEAT_OFF_C0";
      )     ;
      R     "DB_POWER_SAVING_MODE2".MODE.WD1_ASU_HEATING;
      U     L     36.0;
      U     "DB_POWER_SAVING_MODE2".MODE.WD1_ASU_COOLING;
      U     "DB_GRP_81".VA41.SM.Close;
      U(    ;
      L     "DB_GRP_81".CLT81.PV.AV;
      L     #SW_WD1_ASU_STOP_COOLING;
      <R    ;
      )     ;
      L     S5T#40S;
      SE    "T_PS_M2_WD1_COOL_OFF_C0";
      NOP   0;
      NOP   0;
      NOP   0;
      NOP   0;
      U     L     36.0;
      U(    ;
      L     "DB_GRP_81".CLT81.PV.AV;
      L     "DB_POWER_SAVING_MODE2".GENERAL.SP.WD1_ASU_WINDOW_T_MAX;
      >R    ;
      )     ;
      S     "DB_POWER_SAVING_MODE2".MODE.WD1_ASU_COOLING;
      U     L     36.0;
      U(    ;
      O     "DB_POWER_SAVING_MODE2".MODE.WD1_ASU_HEATING;
      O     "T_PS_M2_WD1_COOL_OFF_C0";
      )     ;
      R     "DB_POWER_SAVING_MODE2".MODE.WD1_ASU_COOLING;
      U     L     36.0;
      U     "DB_POWER_SAVING_MODE2".MODE.WD1_ASU_COOLING;
      SPBNB _01d;
      L     "DB_POWER_SAVING_MODE2".GENERAL.SP.WD1_ASU_WINDOW_T_MAX;
      T     "DB_POWER_SAVING_MODE2".GENERAL.SP.WD1_ASU_T;
_01d: NOP   0;
      U     L     36.0;
      U     "DB_POWER_SAVING_MODE2".MODE.WD1_ASU_HEATING;
      SPBNB _01e;
      L     "DB_POWER_SAVING_MODE2".GENERAL.SP.WD1_ASU_WINDOW_T_MIN;
      T     "DB_POWER_SAVING_MODE2".GENERAL.SP.WD1_ASU_T;
_01e: NOP   0;
      U     L     36.0;
      UN    "DB_POWER_SAVING_MODE2".MODE.WD1_ASU_COOLING;
      UN    "DB_POWER_SAVING_MODE2".MODE.WD1_ASU_HEATING;
      SPBNB _01f;
      L     "DB_GRP_81".CLT81.PV.AV;
      T     "DB_POWER_SAVING_MODE2".GENERAL.SP.WD1_ASU_T;
_01f: NOP   0;
NETWORK
TITLE =WORKDECK'S 1 CONDITION 1
//OUTSIDE TEMPERATURE < T MIN
//
//HEATING ON
//COOLING OFF
//UNTIL WINDOW IS REACHED
//
//HEATING SP T MIN
      U     "DB_POWER_SAVING_MODE2".CONDITIONS.WD1_C1;
      =     L     36.0;
      U     L     36.0;
      BLD   102;
      R     "DB_POWER_SAVING_MODE2".MODE.WD1_ASU_COOLING;
      U     L     36.0;
      U(    ;
      L     "DB_GRP_81".CLT81.PV.AV;
      L     "DB_POWER_SAVING_MODE2".GENERAL.SP.WD1_ASU_WINDOW_T_MIN;
      <R    ;
      )     ;
      S     "DB_POWER_SAVING_MODE2".MODE.WD1_ASU_HEATING;
      U     L     36.0;
      U     "DB_POWER_SAVING_MODE2".MODE.WD1_ASU_HEATING;
      U     "DB_GRP_81".VA31.SM.Open;
      U(    ;
      L     "DB_GRP_81".PP31.PV.AV;
      L     8.000000e+000;
      <=R   ;
      )     ;
      U(    ;
      L     "DB_GRP_81".CLT81.PV.AV;
      L     #SW_WD1_ASU_STOP_HEATING;
      >R    ;
      )     ;
      L     S5T#40S;
      SE    "T_PS_M2_WD1_HEAT_OFF_C1";
      NOP   0;
      NOP   0;
      NOP   0;
      U     "T_PS_M2_WD1_HEAT_OFF_C1";
      R     "DB_POWER_SAVING_MODE2".MODE.WD1_ASU_HEATING;
      U     L     36.0;
      U     "DB_POWER_SAVING_MODE2".MODE.WD1_ASU_HEATING;
      SPBNB _020;
      L     "DB_POWER_SAVING_MODE2".GENERAL.SP.WD1_ASU_WINDOW_T_MIN;
      T     "DB_POWER_SAVING_MODE2".GENERAL.SP.WD1_ASU_T;
_020: NOP   0;
      U     L     36.0;
      UN    "DB_POWER_SAVING_MODE2".MODE.WD1_ASU_HEATING;
      SPBNB _021;
      L     "DB_GRP_81".CLT81.PV.AV;
      T     "DB_POWER_SAVING_MODE2".GENERAL.SP.WD1_ASU_T;
_021: NOP   0;
NETWORK
TITLE =WORKDECK'S 1 CONDITION 2
//OUTSIDE TEMPERATURE > T MAX
//
//HEATING OFF
//COOLING ON
//UNTIL WINDOW IS REACHED
//
//COOLING SP T MAX
      U     "DB_POWER_SAVING_MODE2".CONDITIONS.WD1_C2;
      =     L     36.0;
      U     L     36.0;
      U(    ;
      L     "DB_GRP_81".CLT81.PV.AV;
      L     "DB_POWER_SAVING_MODE2".GENERAL.SP.WD1_ASU_WINDOW_T_MAX;
      >R    ;
      )     ;
      S     "DB_POWER_SAVING_MODE2".MODE.WD1_ASU_COOLING;
      U     L     36.0;
      U     "DB_POWER_SAVING_MODE2".MODE.WD1_ASU_COOLING;
      U     "DB_GRP_81".VA41.SM.Close;
      U(    ;
      L     "DB_GRP_81".CLT81.PV.AV;
      L     #SW_WD1_ASU_STOP_COOLING;
      <R    ;
      )     ;
      L     S5T#1M;
      SE    "T_PS_M2_WD1_COOL_OFF_C2";
      NOP   0;
      NOP   0;
      NOP   0;
      U     "T_PS_M2_WD1_COOL_OFF_C2";
      R     "DB_POWER_SAVING_MODE2".MODE.WD1_ASU_COOLING;
      U     L     36.0;
      BLD   102;
      R     "DB_POWER_SAVING_MODE2".MODE.WD1_ASU_HEATING;
      U     L     36.0;
      U     "DB_POWER_SAVING_MODE2".MODE.WD1_ASU_COOLING;
      SPBNB _022;
      L     "DB_POWER_SAVING_MODE2".GENERAL.SP.WD1_ASU_WINDOW_T_MAX;
      T     "DB_POWER_SAVING_MODE2".GENERAL.SP.WD1_ASU_T;
_022: NOP   0;
      U     L     36.0;
      UN    "DB_POWER_SAVING_MODE2".MODE.WD1_ASU_COOLING;
      SPBNB _023;
      L     "DB_GRP_81".CLT81.PV.AV;
      T     "DB_POWER_SAVING_MODE2".GENERAL.SP.WD1_ASU_T;
_023: NOP   0;
NETWORK
TITLE =TRANSFER SETPOINTS FOR WORKDECK'S 1
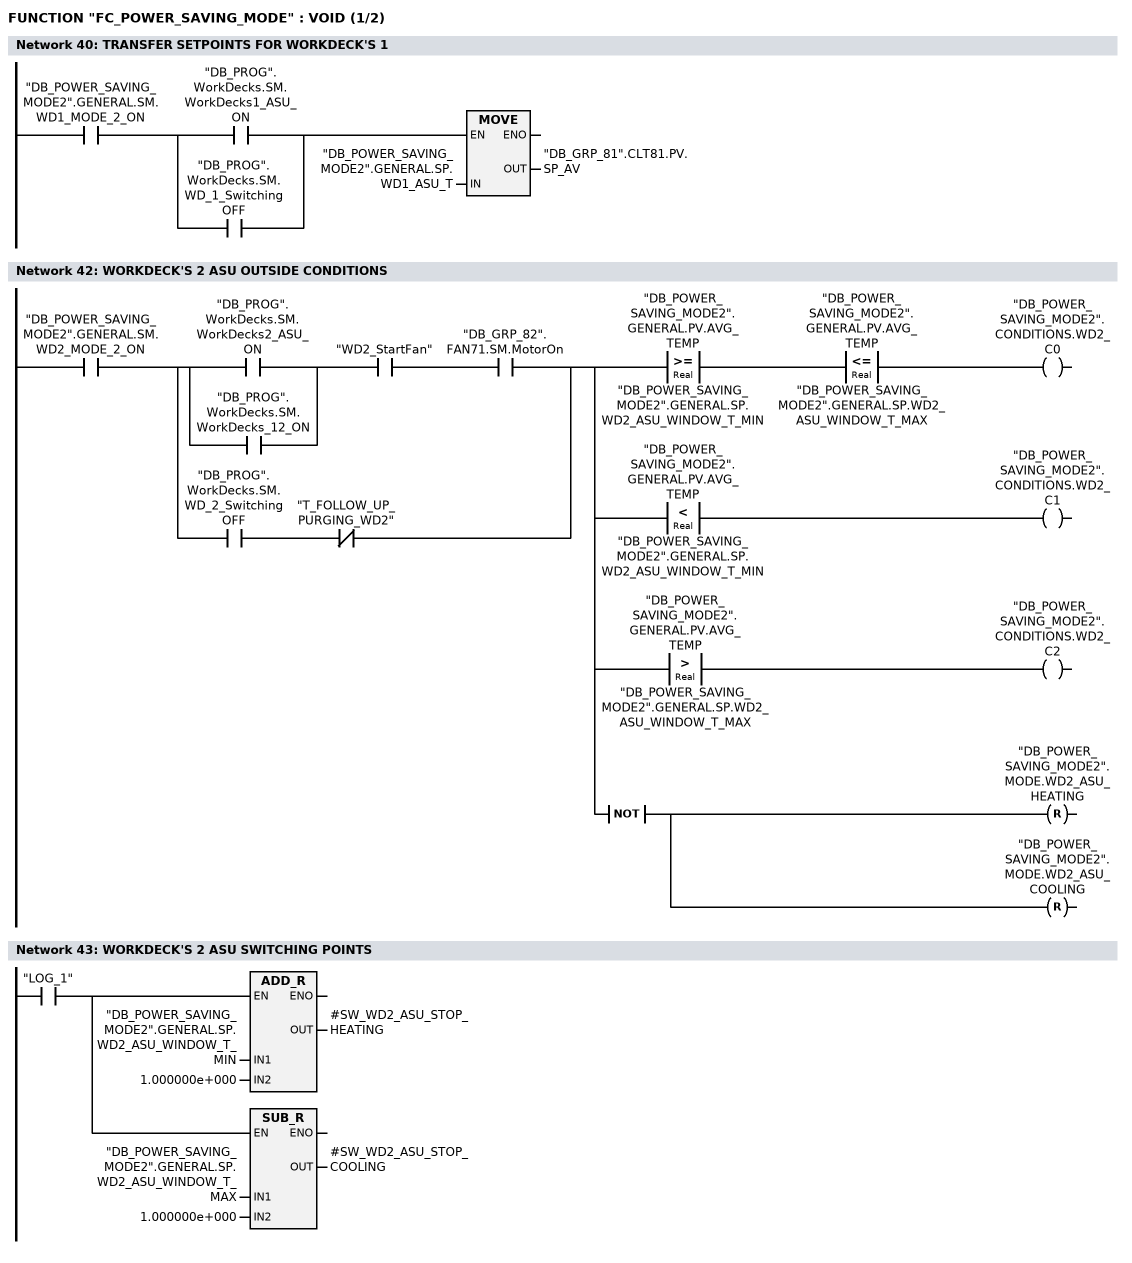
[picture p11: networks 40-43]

      U     "DB_POWER_SAVING_MODE2".GENERAL.SM.WD1_MODE_2_ON;
      U(    ;
      O     "DB_PROG".WorkDecks.SM.WorkDecks1_ASU_ON;
      O     "DB_PROG".WorkDecks.SM.WD_1_SwitchingOFF;
      )     ;
      SPBNB _024;
      L     "DB_POWER_SAVING_MODE2".GENERAL.SP.WD1_ASU_T;
      T     "DB_GRP_81".CLT81.PV.SP_AV;
_024: NOP   0;
NETWORK
TITLE =************** START ECO MODE 2 WORKDECK'S 2 *************

NETWORK
TITLE =WORKDECK'S 2 ASU OUTSIDE CONDITIONS

      U     "DB_POWER_SAVING_MODE2".GENERAL.SM.WD2_MODE_2_ON;
      U(    ;
      U(    ;
      O     "DB_PROG".WorkDecks.SM.WorkDecks2_ASU_ON;
      O     "DB_PROG".WorkDecks.SM.WorkDecks_12_ON;
      )     ;
      U     "WD2_StartFan";
      U     "DB_GRP_82".FAN71.SM.MotorOn;
      O     ;
      U     "DB_PROG".WorkDecks.SM.WD_2_SwitchingOFF;
      UN    "T_FOLLOW_UP_PURGING_WD2";
      )     ;
      =     L     36.0;
      U     L     36.0;
      U(    ;
      L     "DB_POWER_SAVING_MODE2".GENERAL.PV.AVG_TEMP;
      L     "DB_POWER_SAVING_MODE2".GENERAL.SP.WD2_ASU_WINDOW_T_MIN;
      >=R   ;
      )     ;
      U(    ;
      L     "DB_POWER_SAVING_MODE2".GENERAL.PV.AVG_TEMP;
      L     "DB_POWER_SAVING_MODE2".GENERAL.SP.WD2_ASU_WINDOW_T_MAX;
      <=R   ;
      )     ;
      =     "DB_POWER_SAVING_MODE2".CONDITIONS.WD2_C0;
      U     L     36.0;
      U(    ;
      L     "DB_POWER_SAVING_MODE2".GENERAL.PV.AVG_TEMP;
      L     "DB_POWER_SAVING_MODE2".GENERAL.SP.WD2_ASU_WINDOW_T_MIN;
      <R    ;
      )     ;
      =     "DB_POWER_SAVING_MODE2".CONDITIONS.WD2_C1;
      U     L     36.0;
      U(    ;
      L     "DB_POWER_SAVING_MODE2".GENERAL.PV.AVG_TEMP;
      L     "DB_POWER_SAVING_MODE2".GENERAL.SP.WD2_ASU_WINDOW_T_MAX;
      >R    ;
      )     ;
      =     "DB_POWER_SAVING_MODE2".CONDITIONS.WD2_C2;
      U     L     36.0;
      NOT   ;
      R     "DB_POWER_SAVING_MODE2".MODE.WD2_ASU_HEATING;
      R     "DB_POWER_SAVING_MODE2".MODE.WD2_ASU_COOLING;
NETWORK
TITLE =WORKDECK'S 2 ASU SWITCHING POINTS

      U     "LOG_1";
      =     L     36.0;
      U     L     36.0;
      SPBNB _025;
      L     "DB_POWER_SAVING_MODE2".GENERAL.SP.WD2_ASU_WINDOW_T_MIN;
      L     1.000000e+000;
      +R    ;
      T     #SW_WD2_ASU_STOP_HEATING;
_025: NOP   0;
      U     L     36.0;
      SPBNB _026;
      L     "DB_POWER_SAVING_MODE2".GENERAL.SP.WD2_ASU_WINDOW_T_MAX;
      L     1.000000e+000;
      -R    ;
      T     #SW_WD2_ASU_STOP_COOLING;
_026: NOP   0;
NETWORK
TITLE =WORKDECK'S 2 CONDIDITON 0
//OUTSIDE TEMPERATURE IN WINDOW
//
//HEATING OFF
//COOLING OFF
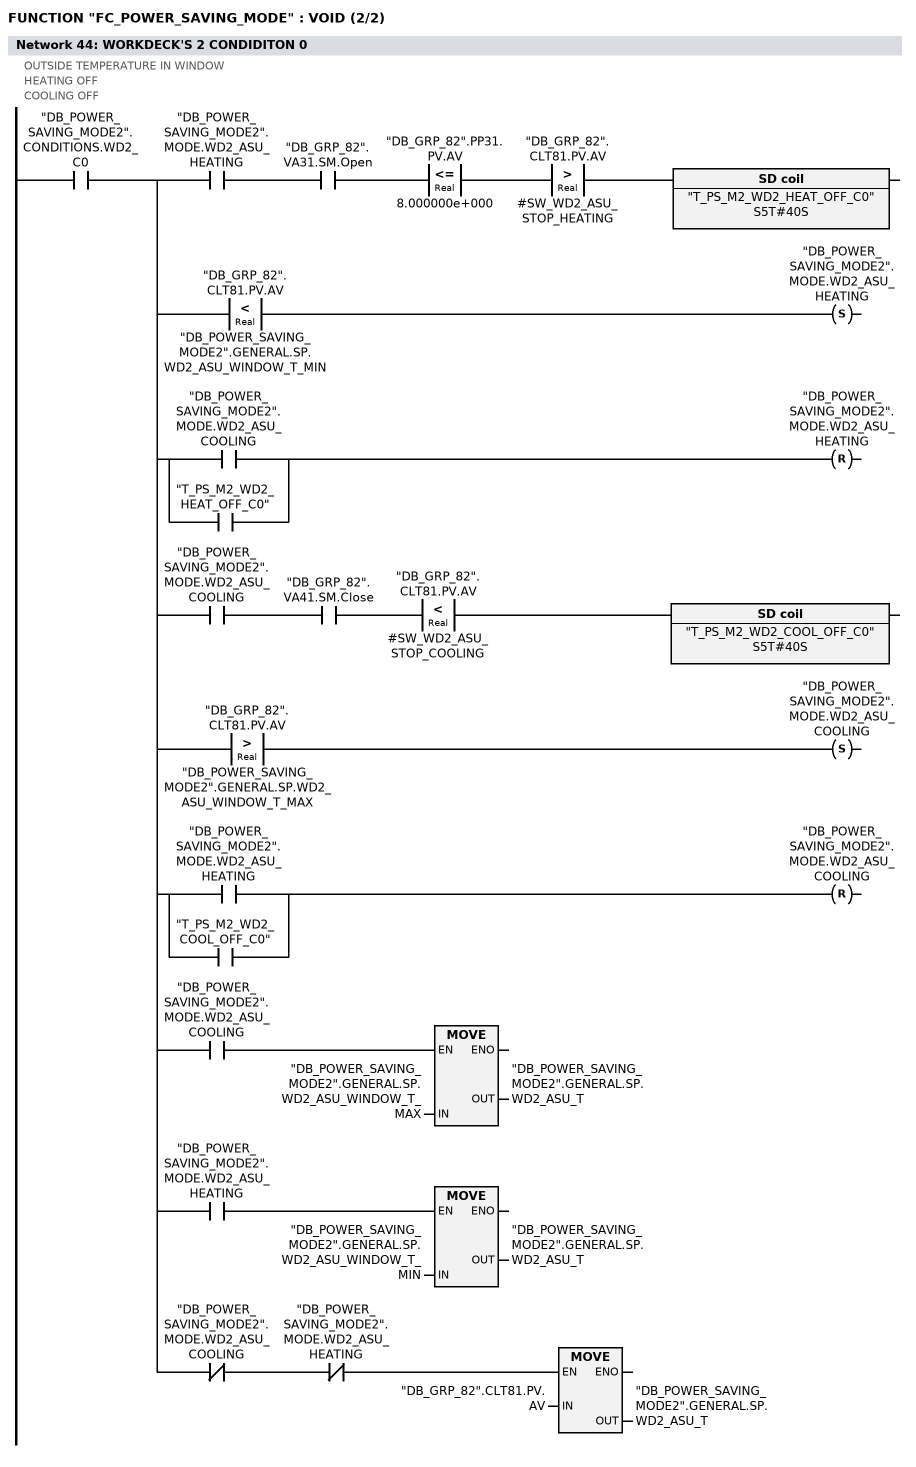
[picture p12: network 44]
      U     "DB_POWER_SAVING_MODE2".CONDITIONS.WD2_C0;
      =     L     36.0;
      U     L     36.0;
      U     "DB_POWER_SAVING_MODE2".MODE.WD2_ASU_HEATING;
      U     "DB_GRP_82".VA31.SM.Open;
      U(    ;
      L     "DB_GRP_82".PP31.PV.AV;
      L     8.000000e+000;
      <=R   ;
      )     ;
      U(    ;
      L     "DB_GRP_82".CLT81.PV.AV;
      L     #SW_WD2_ASU_STOP_HEATING;
      >R    ;
      )     ;
      L     S5T#40S;
      SE    "T_PS_M2_WD2_HEAT_OFF_C0";
      NOP   0;
      NOP   0;
      NOP   0;
      NOP   0;
      U     L     36.0;
      U(    ;
      L     "DB_GRP_82".CLT81.PV.AV;
      L     "DB_POWER_SAVING_MODE2".GENERAL.SP.WD2_ASU_WINDOW_T_MIN;
      <R    ;
      )     ;
      S     "DB_POWER_SAVING_MODE2".MODE.WD2_ASU_HEATING;
      U     L     36.0;
      U(    ;
      O     "DB_POWER_SAVING_MODE2".MODE.WD2_ASU_COOLING;
      O     "T_PS_M2_WD2_HEAT_OFF_C0";
      )     ;
      R     "DB_POWER_SAVING_MODE2".MODE.WD2_ASU_HEATING;
      U     L     36.0;
      U     "DB_POWER_SAVING_MODE2".MODE.WD2_ASU_COOLING;
      U     "DB_GRP_82".VA41.SM.Close;
      U(    ;
      L     "DB_GRP_82".CLT81.PV.AV;
      L     #SW_WD2_ASU_STOP_COOLING;
      <R    ;
      )     ;
      L     S5T#40S;
      SE    "T_PS_M2_WD2_COOL_OFF_C0";
      NOP   0;
      NOP   0;
      NOP   0;
      NOP   0;
      U     L     36.0;
      U(    ;
      L     "DB_GRP_82".CLT81.PV.AV;
      L     "DB_POWER_SAVING_MODE2".GENERAL.SP.WD2_ASU_WINDOW_T_MAX;
      >R    ;
      )     ;
      S     "DB_POWER_SAVING_MODE2".MODE.WD2_ASU_COOLING;
      U     L     36.0;
      U(    ;
      O     "DB_POWER_SAVING_MODE2".MODE.WD2_ASU_HEATING;
      O     "T_PS_M2_WD2_COOL_OFF_C0";
      )     ;
      R     "DB_POWER_SAVING_MODE2".MODE.WD2_ASU_COOLING;
      U     L     36.0;
      U     "DB_POWER_SAVING_MODE2".MODE.WD2_ASU_COOLING;
      SPBNB _027;
      L     "DB_POWER_SAVING_MODE2".GENERAL.SP.WD2_ASU_WINDOW_T_MAX;
      T     "DB_POWER_SAVING_MODE2".GENERAL.SP.WD2_ASU_T;
_027: NOP   0;
      U     L     36.0;
      U     "DB_POWER_SAVING_MODE2".MODE.WD2_ASU_HEATING;
      SPBNB _028;
      L     "DB_POWER_SAVING_MODE2".GENERAL.SP.WD2_ASU_WINDOW_T_MIN;
      T     "DB_POWER_SAVING_MODE2".GENERAL.SP.WD2_ASU_T;
_028: NOP   0;
      U     L     36.0;
      UN    "DB_POWER_SAVING_MODE2".MODE.WD2_ASU_COOLING;
      UN    "DB_POWER_SAVING_MODE2".MODE.WD2_ASU_HEATING;
      SPBNB _029;
      L     "DB_GRP_82".CLT81.PV.AV;
      T     "DB_POWER_SAVING_MODE2".GENERAL.SP.WD2_ASU_T;
_029: NOP   0;
NETWORK
TITLE =WORKDECK'S 2 CONDITION 1
//OUTSIDE TEMPERATURE < T MIN
//
//HEATING ON
//COOLING OFF
//UNTIL WINDOW IS REACHED
//
//HEATING SP T MIN
      U     "DB_POWER_SAVING_MODE2".CONDITIONS.WD2_C1;
      =     L     36.0;
      U     L     36.0;
      BLD   102;
      R     "DB_POWER_SAVING_MODE2".MODE.WD2_ASU_COOLING;
      U     L     36.0;
      U(    ;
      L     "DB_GRP_82".CLT81.PV.AV;
      L     "DB_POWER_SAVING_MODE2".GENERAL.SP.WD2_ASU_WINDOW_T_MIN;
      <R    ;
      )     ;
      S     "DB_POWER_SAVING_MODE2".MODE.WD2_ASU_HEATING;
      U     L     36.0;
      U     "DB_POWER_SAVING_MODE2".MODE.WD2_ASU_HEATING;
      U     "DB_GRP_82".VA31.SM.Open;
      U(    ;
      L     "DB_GRP_82".PP31.PV.AV;
      L     8.000000e+000;
      <=R   ;
      )     ;
      U(    ;
      L     "DB_GRP_82".CLT81.PV.AV;
      L     #SW_WD2_ASU_STOP_HEATING;
      >R    ;
      )     ;
      L     S5T#40S;
      SE    "T_PS_M2_WD2_HEAT_OFF_C1";
      NOP   0;
      NOP   0;
      NOP   0;
      U     "T_PS_M2_WD2_HEAT_OFF_C1";
      R     "DB_POWER_SAVING_MODE2".MODE.WD2_ASU_HEATING;
      U     L     36.0;
      U     "DB_POWER_SAVING_MODE2".MODE.WD2_ASU_HEATING;
      SPBNB _02a;
      L     "DB_POWER_SAVING_MODE2".GENERAL.SP.WD2_ASU_WINDOW_T_MIN;
      T     "DB_POWER_SAVING_MODE2".GENERAL.SP.WD2_ASU_T;
_02a: NOP   0;
      U     L     36.0;
      UN    "DB_POWER_SAVING_MODE2".MODE.WD2_ASU_HEATING;
      SPBNB _02b;
      L     "DB_GRP_82".CLT81.PV.AV;
      T     "DB_POWER_SAVING_MODE2".GENERAL.SP.WD2_ASU_T;
_02b: NOP   0;
NETWORK
TITLE =WORKDECK'S 2 CONDITION 2
//OUTSIDE TEMPERATURE > T MAX
//
//HEATING OFF
//COOLING ON
//UNTIL WINDOW IS REACHED
//
//COOLING SP T MAX
      U     "DB_POWER_SAVING_MODE2".CONDITIONS.WD2_C2;
      =     L     36.0;
      U     L     36.0;
      U(    ;
      L     "DB_GRP_82".CLT81.PV.AV;
      L     "DB_POWER_SAVING_MODE2".GENERAL.SP.WD2_ASU_WINDOW_T_MAX;
      >R    ;
      )     ;
      S     "DB_POWER_SAVING_MODE2".MODE.WD2_ASU_COOLING;
      U     L     36.0;
      U     "DB_POWER_SAVING_MODE2".MODE.WD2_ASU_COOLING;
      U     "DB_GRP_82".VA41.SM.Close;
      U(    ;
      L     "DB_GRP_82".CLT81.PV.AV;
      L     #SW_WD2_ASU_STOP_COOLING;
      <R    ;
      )     ;
      L     S5T#1M;
      SE    "T_PS_M2_WD2_COOL_OFF_C2";
      NOP   0;
      NOP   0;
      NOP   0;
      U     "T_PS_M2_WD2_COOL_OFF_C2";
      R     "DB_POWER_SAVING_MODE2".MODE.WD2_ASU_COOLING;
      U     L     36.0;
      BLD   102;
      R     "DB_POWER_SAVING_MODE2".MODE.WD2_ASU_HEATING;
      U     L     36.0;
      U     "DB_POWER_SAVING_MODE2".MODE.WD2_ASU_COOLING;
      SPBNB _02c;
      L     "DB_POWER_SAVING_MODE2".GENERAL.SP.WD2_ASU_WINDOW_T_MAX;
      T     "DB_POWER_SAVING_MODE2".GENERAL.SP.WD2_ASU_T;
_02c: NOP   0;
      U     L     36.0;
      UN    "DB_POWER_SAVING_MODE2".MODE.WD2_ASU_COOLING;
      SPBNB _02d;
      L     "DB_GRP_82".CLT81.PV.AV;
      T     "DB_POWER_SAVING_MODE2".GENERAL.SP.WD2_ASU_T;
_02d: NOP   0;
NETWORK
TITLE =TRANSFER SETPOINTS FOR WORKDECK'S 2
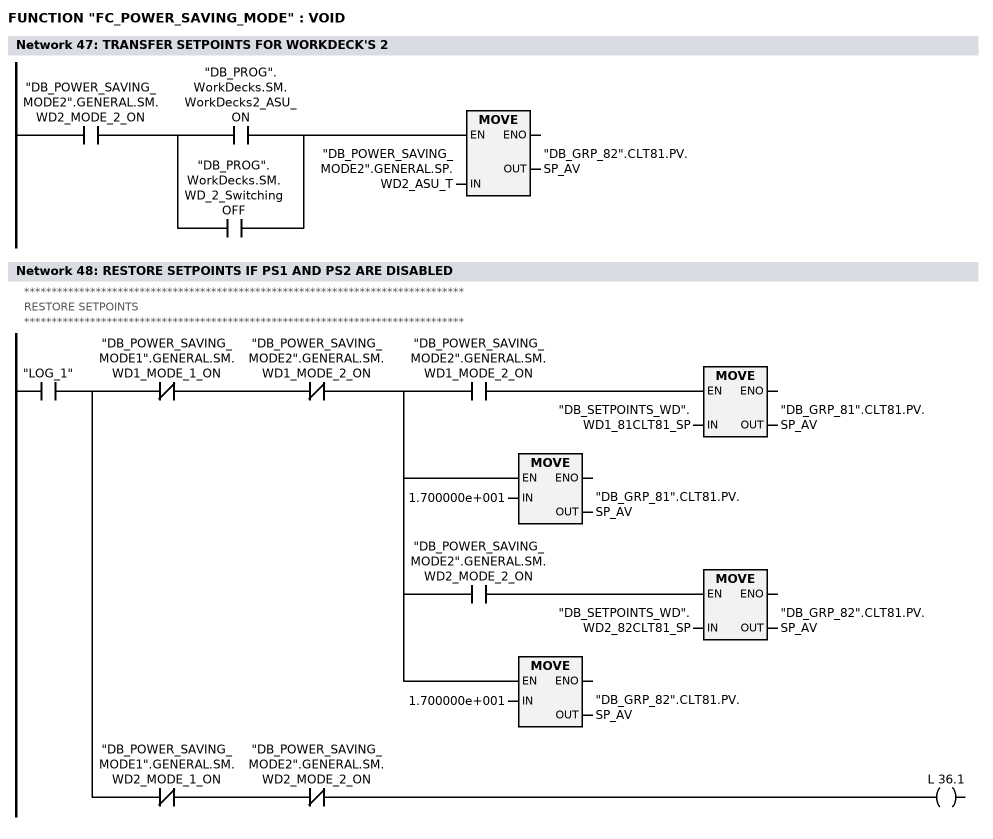
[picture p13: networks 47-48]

      U     "DB_POWER_SAVING_MODE2".GENERAL.SM.WD2_MODE_2_ON;
      U(    ;
      O     "DB_PROG".WorkDecks.SM.WorkDecks2_ASU_ON;
      O     "DB_PROG".WorkDecks.SM.WD_2_SwitchingOFF;
      )     ;
      SPBNB _02e;
      L     "DB_POWER_SAVING_MODE2".GENERAL.SP.WD2_ASU_T;
      T     "DB_GRP_82".CLT81.PV.SP_AV;
_02e: NOP   0;
NETWORK
TITLE =RESTORE SETPOINTS IF PS1 AND PS2 ARE DISABLED
//********************************************************************************
//
//                               RESTORE SETPOINTS
//
//********************************************************************************
//
      U     "LOG_1";
      =     L     36.0;
      U     L     36.0;
      UN    "DB_POWER_SAVING_MODE1".GENERAL.SM.WD1_MODE_1_ON;
      UN    "DB_POWER_SAVING_MODE2".GENERAL.SM.WD1_MODE_2_ON;
      =     L     36.1;
      U     L     36.1;
      U     "DB_POWER_SAVING_MODE2".GENERAL.SM.WD1_MODE_2_ON;
      SPBNB _02f;
      L     "DB_SETPOINTS_WD".WD1_81CLT81_SP;
      T     "DB_GRP_81".CLT81.PV.SP_AV;
_02f: NOP   0;
      U     L     36.1;
      SPBNB _030;
      L     1.700000e+001;
      T     "DB_GRP_81".CLT81.PV.SP_AV;
_030: NOP   0;
      U     L     36.0;
      UN    "DB_POWER_SAVING_MODE1".GENERAL.SM.WD2_MODE_1_ON;
      UN    "DB_POWER_SAVING_MODE2".GENERAL.SM.WD2_MODE_2_ON;
      =     L     36.1;
      U     L     36.1;
      U     "DB_POWER_SAVING_MODE2".GENERAL.SM.WD2_MODE_2_ON;
      SPBNB _031;
      L     "DB_SETPOINTS_WD".WD2_82CLT81_SP;
      T     "DB_GRP_82".CLT81.PV.SP_AV;
_031: NOP   0;
      U     L     36.1;
      SPBNB _032;
      L     1.700000e+001;
      T     "DB_GRP_82".CLT81.PV.SP_AV;
_032: NOP   0;
END_FUNCTION

